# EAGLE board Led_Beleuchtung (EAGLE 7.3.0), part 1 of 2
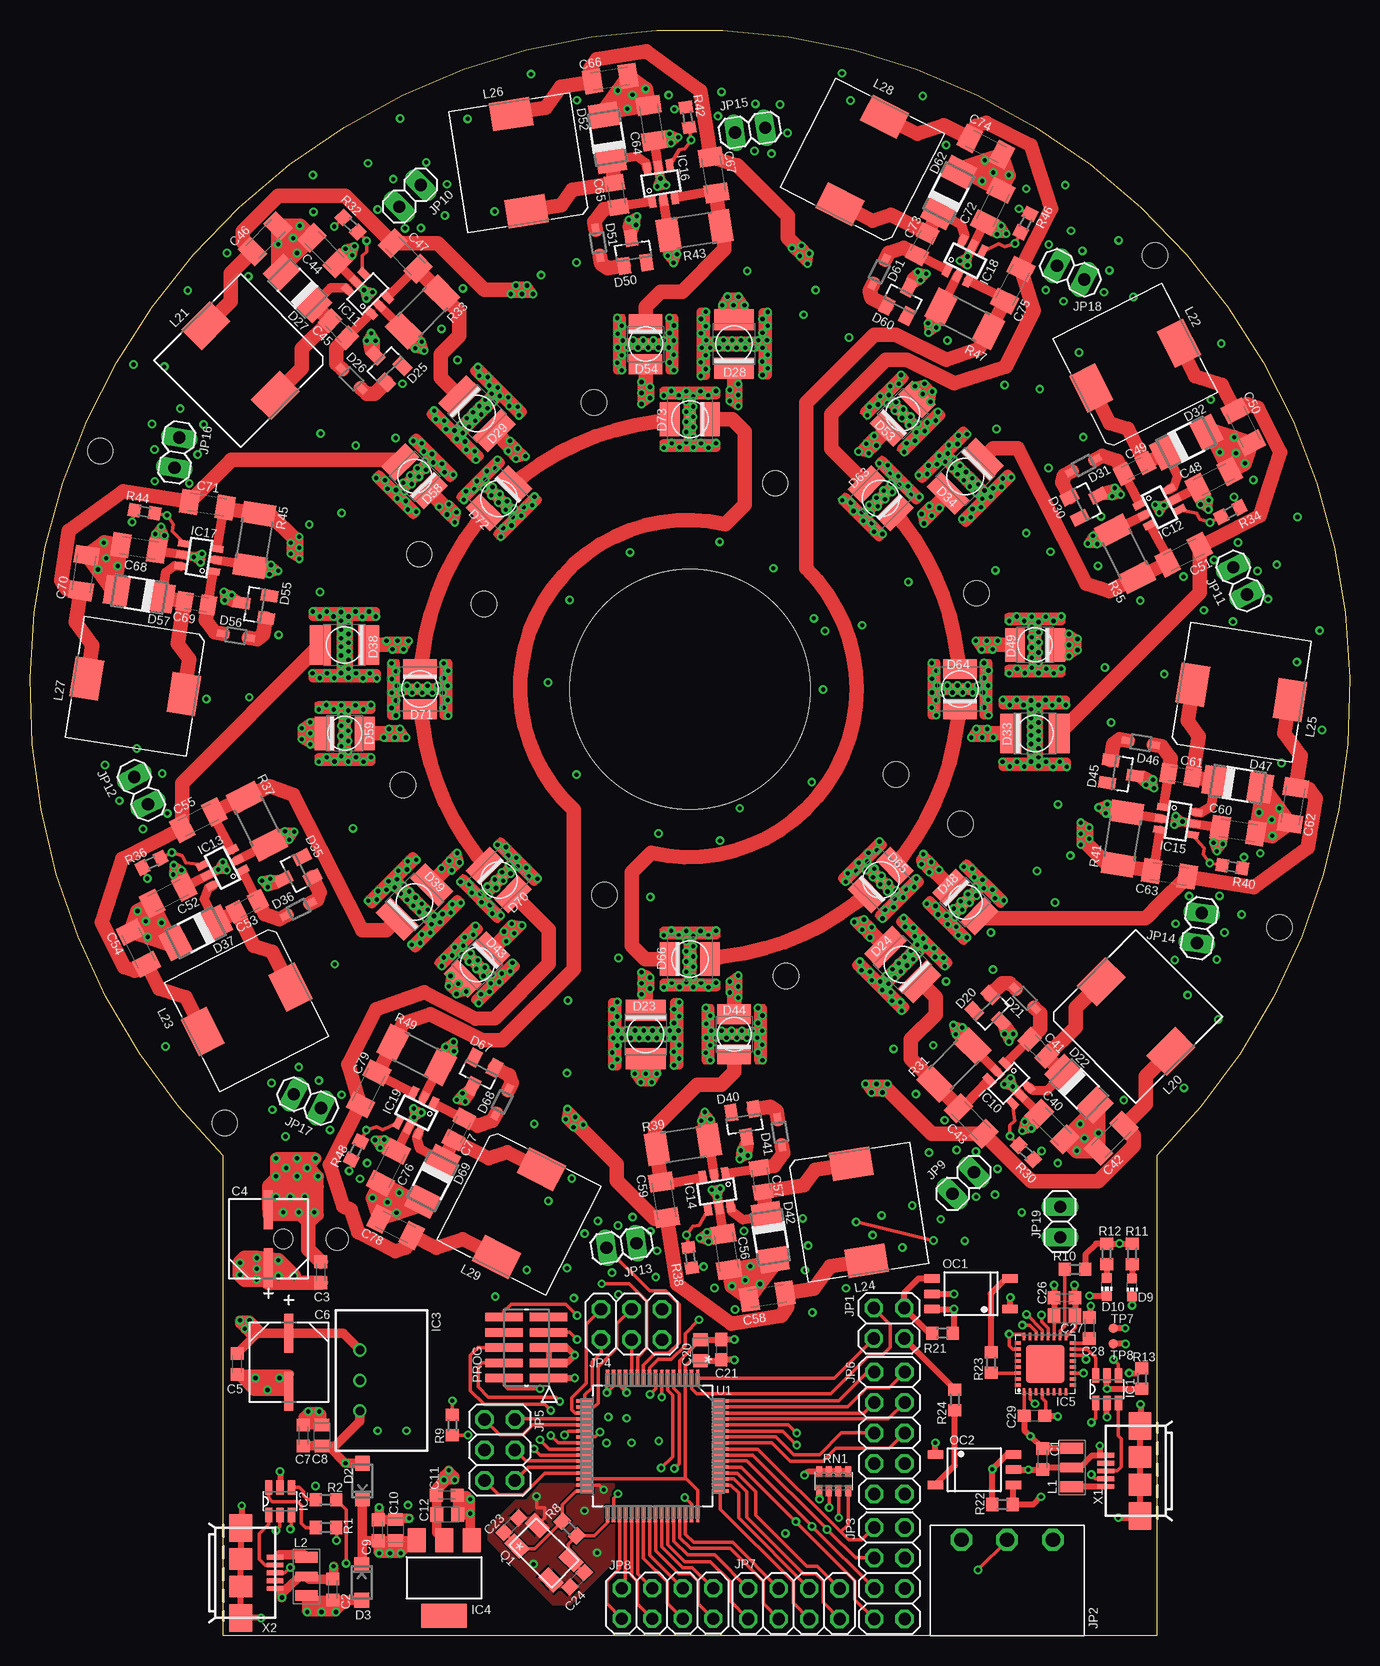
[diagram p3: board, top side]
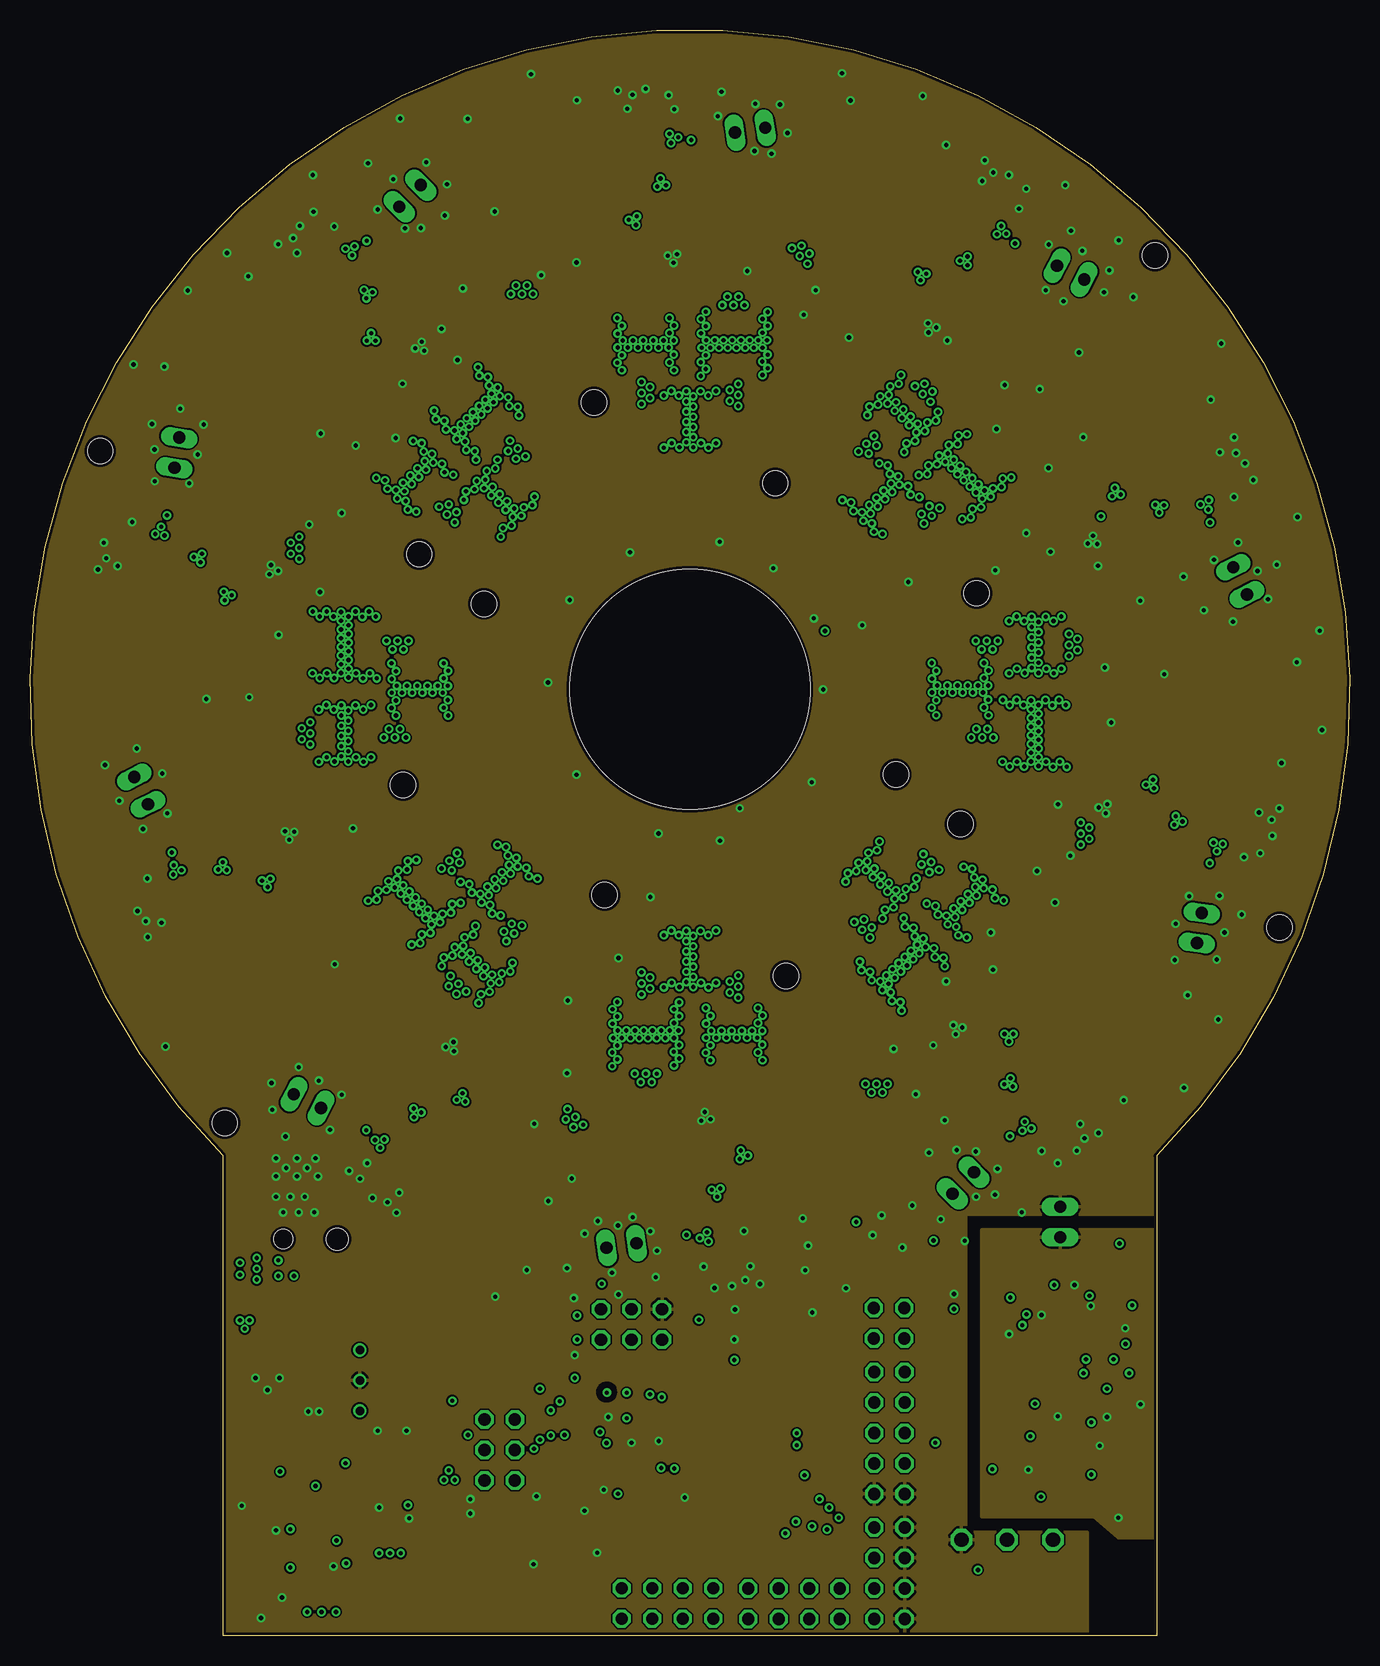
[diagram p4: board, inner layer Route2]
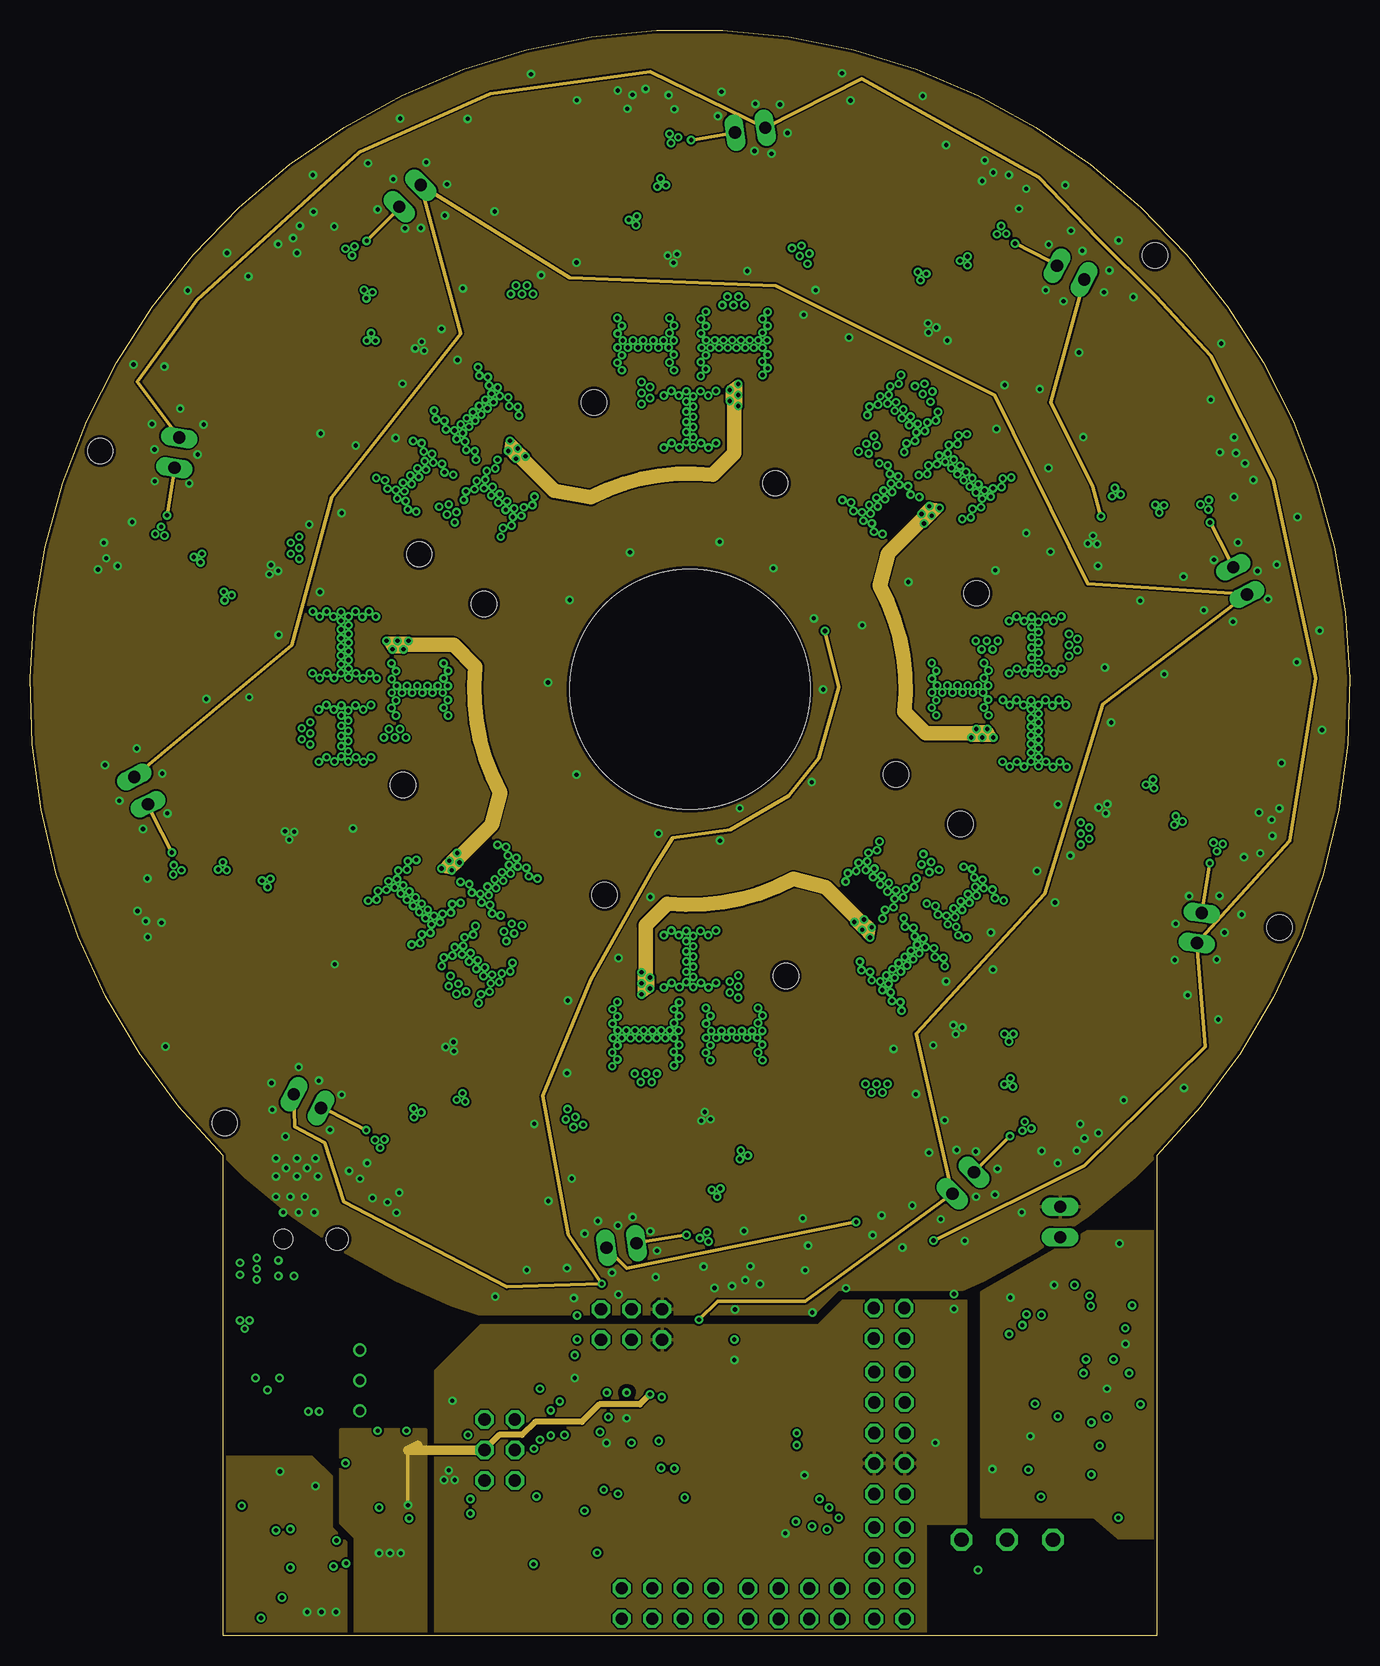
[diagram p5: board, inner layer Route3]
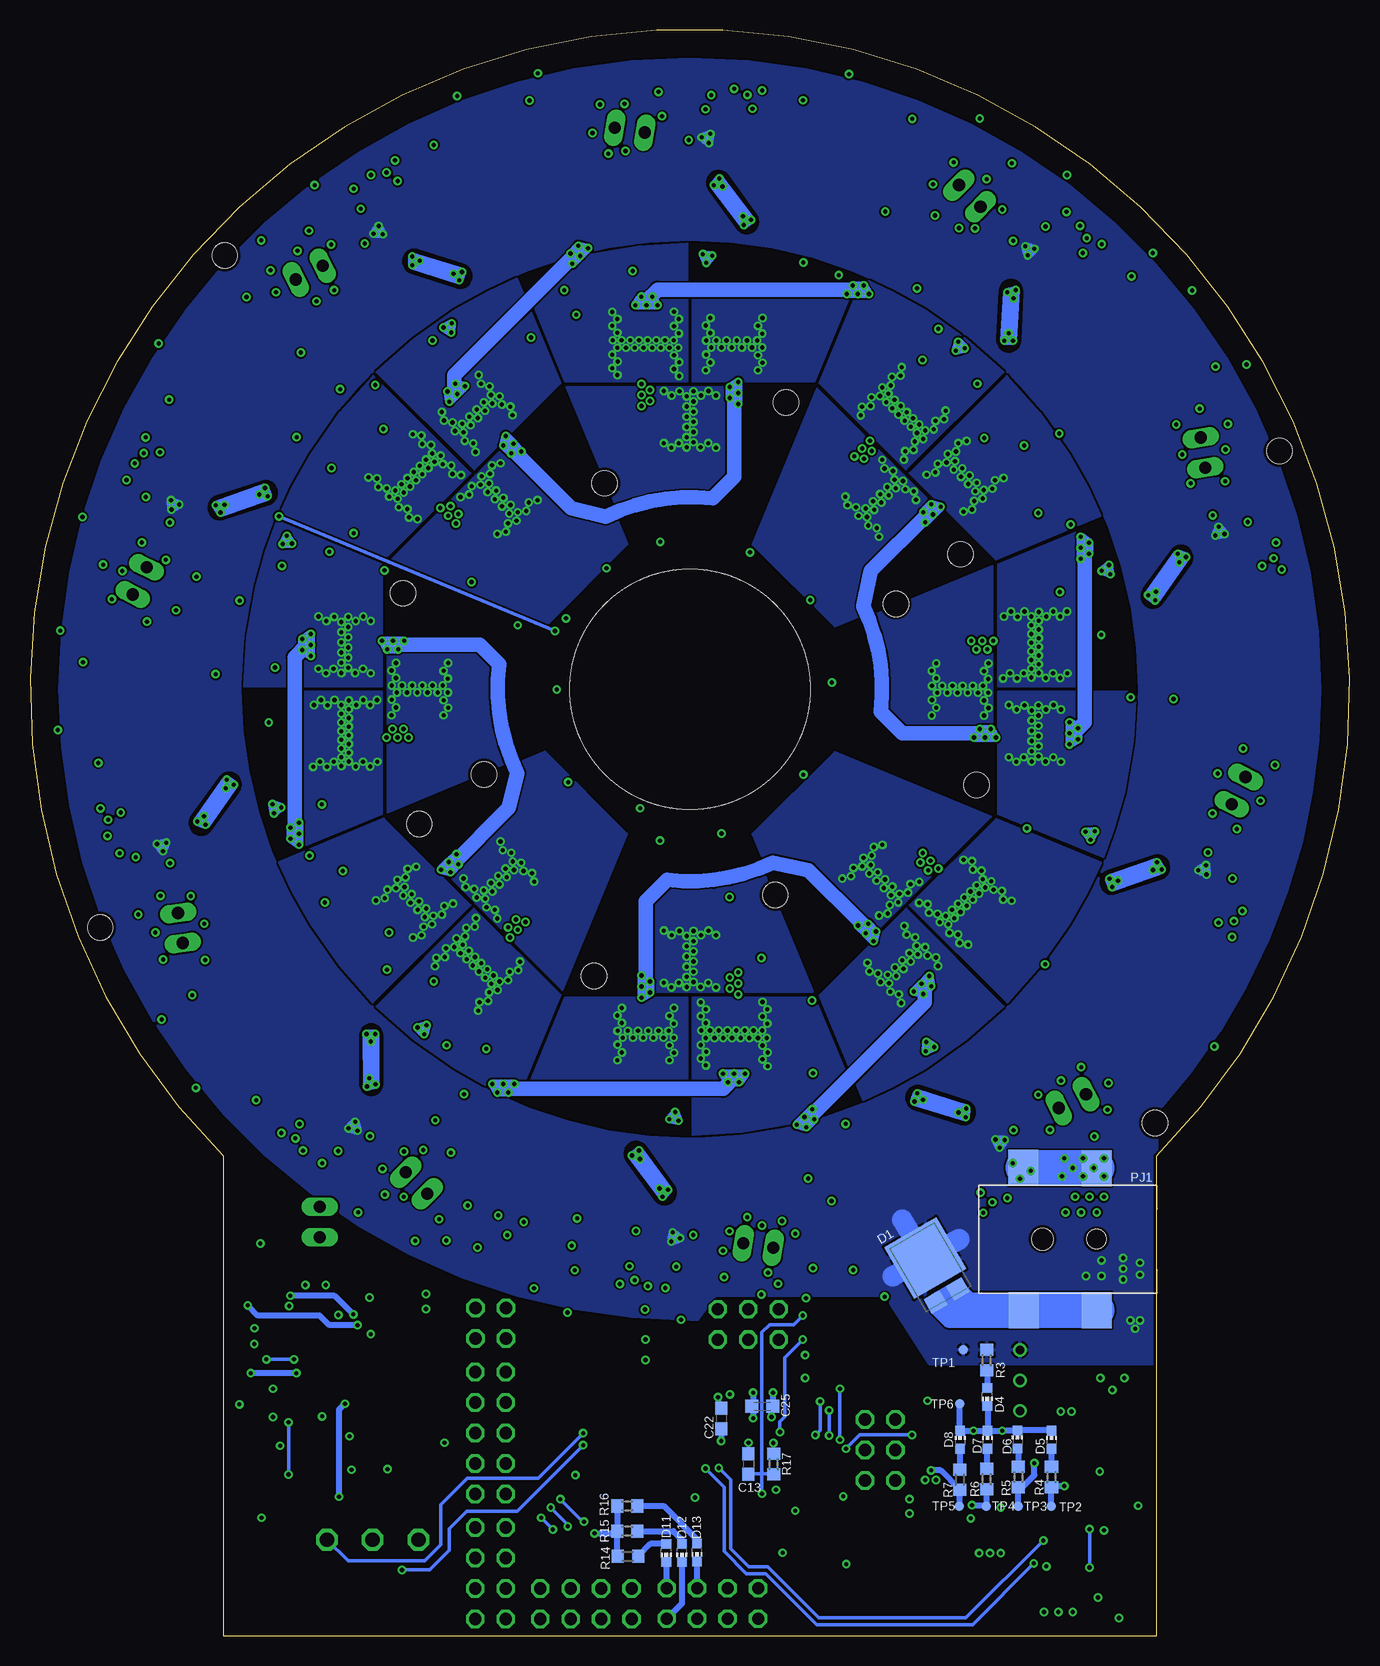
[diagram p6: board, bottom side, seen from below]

Size 109.98 x 133.82 mm. Coordinates in mm from the lower left corner, seen from the top.
Outline: 16.1,0 16.1,39.99 arc-270 93.88,39.99 93.88,0 16.1,0
Copper layers (1+2*3+16): Top 0.018mm / dielectric 0.36mm / Route2 0.035mm / dielectric 0.71mm / Route3 0.035mm / dielectric 0.36mm / Bottom 0.018mm
Design rules "eC_4Layer_PClass6_BaseCopperO18-I35_eCDefault *": minimum track width 0.15mm, minimum drill 0.35mm, track to track 0.15mm, track to pad 0.15mm, pad to pad 0.15mm, via to via 0.15mm, smd to smd 0mil, copper to edge 0.25mm, drill to drill 0.35mm, minimum pad ring 0.175mm, minimum via ring 0.125mm, stop-mask expansion 0mil, vias tented up to drill 0.45mm, thermal gap 0.2mm
Holes 2.1 mm at 62.1,96.05 37.83,85.99 47.88,61.72 72.15,71.78 32.44,90.13 47,102.78 78.89,86.88 77.54,67.64 62.99,54.99 31.09,70.89 5.85,98.74 93.75,115.03 104.13,59.03 16.23,42.74
Holes 20 mm at 54.99,78.88

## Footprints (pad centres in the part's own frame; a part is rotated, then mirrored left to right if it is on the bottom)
C0603K = smd 1.05 x 1.08: 1 -0.875,0; 2 0.875,0
CAPAE660X800N = smd 3.251 x 0.762: 1 -2.413,0; 2 2.413,0
CAPAE660X610N = smd 3.251 x 0.762: 1 -2.413,0; 2 2.413,0
SMC_P = smd 1.05 x 1.2: + -0.875,0; - 0.875,0
C0603 = smd 1.1 x 1: 1 -0.85,0; 2 0.85,0
C1206K = smd 1.5 x 2: 1 -1.5,0; 2 1.5,0
C0805K = smd 1.3 x 1.6: 1 -1,0; 2 1,0
TO-277A = smd 1.5 x 1.4: A1 1.065,-2.705; A2 -1.065,-2.705 | smd 5 x 5: C 0,0.895
SOD-123 = smd 1.25 x 1.22: A 1.475,0; C -1.475,0
CHIP-LED0603 = smd 0.8 x 0.8: A 0,-0.75; C 0,0.75
SOT23 = smd 1 x 1.4: 1 -0.95,-1.1; 2 0.95,-1.1; 3 0,1.1
SOD323 = smd 1 x 0.6: A 1.1,0; C -1.1,0
DO-214AC = smd 2 x 2.4: A 1.9,0; C -1.9,0
LTPL-C034UVH = smd 3.3 x 1.75: A 0,2.025; C 0,-2.025 | smd 1.27 x 0.635: TH 0,0
GW_CSSRM2.PM = smd 2.8 x 1.65: A 0,1.675; C 0,-1.675 | smd 1.27 x 0.635: TH 0,0
SFH_4715 = smd 2.8 x 1.65: A 0,1.675; C 0,-1.675 | smd 1.27 x 0.635: TH 0,0
SOT-23-6L = smd 0.6 x 1.2: 1 -0.95,-1.15; 2 0,-1.15; 3 0.95,-1.15; 4 0.95,1.15; 5 0,1.15; 6 -0.95,1.15
TSR-1 = drill 0.7 pad 1.1: 1 -2.54,0; 2 0,0; 3 2.54,0
SOT223 = smd 1.5 x 2: 1 -2.3,-3.15; 2 0,-3.15; 3 2.3,-3.15 | smd 3.8 x 2: 4 0,3.15
QFN32 = smd 0.6 x 0.3: 1 -2.3,1.75; 2 -2.3,1.25; 3 -2.3,0.75; 4 -2.3,0.25; 5 -2.3,-0.25; 6 -2.3,-0.75; 7 -2.3,-1.25; 8 -2.3,-1.75; 17 2.3,-1.75; 18 2.3,-1.25; 19 2.3,-0.75; 20 2.3,-0.25; 21 2.3,0.25; 22 2.3,0.75; 23 2.3,1.25; 24 2.3,1.75 | smd 0.3 x 0.6: 9 -1.75,-2.3; 10 -1.25,-2.3; 11 -0.75,-2.3; 12 -0.25,-2.3; 13 0.25,-2.3; 14 0.75,-2.3; 15 1.25,-2.3; 16 1.75,-2.3; 25 1.75,2.3; 26 1.25,2.3; 27 0.75,2.3; 28 0.25,2.3; 29 -0.25,2.3; 30 -0.75,2.3; 31 -1.25,2.3; 32 -1.75,2.3 | smd 3.2 x 3.2: EXP 0,0
DDC6_SOT = smd 0.6 x 1.1: 1 -0.95,-1.35; 2 0,-1.35; 3 0.95,-1.35; 4 0.95,1.35; 5 0,1.35; 6 -0.95,1.35
2X02 = drill 1.016 octagon: 1 -1.27,-1.27; 2 -1.27,1.27; 3 1.27,-1.27; 4 1.27,1.27
BCH-381H-3GN = drill 1.2 octagon: 1 3.81,8; 2 0,8; 3 -3.81,8
2X04 = drill 1.016 octagon: 1 -3.81,-1.27; 2 -3.81,1.27; 3 -1.27,-1.27; 4 -1.27,1.27; 5 1.27,-1.27; 6 1.27,1.27; 7 3.81,-1.27; 8 3.81,1.27
2X03 = drill 1.016 octagon: 1 -2.54,-1.27; 2 -2.54,1.27; 3 0,-1.27; 4 0,1.27; 5 2.54,-1.27; 6 2.54,1.27
2X05 = drill 1.016 octagon: 1 -5.08,-1.27; 2 -5.08,1.27; 3 -2.54,-1.27; 4 -2.54,1.27; 5 0,-1.27; 6 0,1.27; 7 2.54,-1.27; 8 2.54,1.27; 9 5.08,-1.27; 10 5.08,1.27
1X02 = drill 1.016 long: 1 -1.27,0; 2 1.27,0
EMIFILTER = smd 0.9 x 1.9: 1 -1.6,0; 3 1.6,0 | smd 0.8 x 1.9: 2 0,0
WE-PDF = smd 3.4 x 2.4: 1 0,4.1; 2 0,-4.1
PC400 = smd 0.7 x 1.3: 1 -1.27,-3.25; 3 1.27,-3.25; 4 1.27,3.25; 5 0,3.25; 6 -1.27,3.25
PJ-002AH-SMT-TR = smd 2.5 x 3: 1.1 5,5.915; 1.2 11.05,5.915; 2 5,-5.915; 3 11.1,-5.965 | hole 1.6: 5,0 | hole 1.8: 9.5,0
SAMTEC_FTS105-01-L-DV = smd 0.711 x 3.124: 1 -2.54,-1.854; 2 -2.54,1.854; 3 -1.27,-1.854; 4 -1.27,1.854; 5 0,-1.854; 6 0,1.854; 7 1.27,-1.854; 8 1.27,1.854; 9 2.54,-1.854; 10 2.54,1.854
ABM3B = smd 1.8 x 1.2: 1 -2,-1.2; 3 2,1.2; GND1 -2,1.2; GND2 2,-1.2
R0603 = smd 1 x 1.1: 1 -0.85,0; 2 0.85,0
R2010 = smd 1.8 x 2.7: 1 -2.2,0; 2 2.2,0
CTS742C083 = smd 0.5 x 0.9: 1 -1.2,-0.8; 2 -0.4,-0.8; 3 0.4,-0.8; 4 1.2,-0.8; 5 1.2,0.8; 6 0.4,0.8; 7 -0.4,0.8; 8 -1.2,0.8
TP08R = smd 0.8 x 0.8: TP 0,0
QFP50P1200X1200X160-64N = smd 1.422 x 0.279: 1 -5.639,3.759; 2 -5.639,3.251; 3 -5.639,2.743; 4 -5.639,2.261; 5 -5.639,1.753; 6 -5.639,1.245; 7 -5.639,0.762; 8 -5.639,0.254; 9 -5.639,-0.254; 10 -5.639,-0.762; 11 -5.639,-1.245; 12 -5.639,-1.753; 13 -5.639,-2.261; 14 -5.639,-2.743; 15 -5.639,-3.251; 16 -5.639,-3.759; 33 5.639,-3.759; 34 5.639,-3.251; 35 5.639,-2.743; 36 5.639,-2.261; 37 5.639,-1.753; 38 5.639,-1.245; 39 5.639,-0.762; 40 5.639,-0.254; 41 5.639,0.254; 42 5.639,0.762; 43 5.639,1.245; 44 5.639,1.753; 45 5.639,2.261; 46 5.639,2.743; 47 5.639,3.251; 48 5.639,3.759 | smd 0.279 x 1.422: 17 -3.759,-5.639; 18 -3.251,-5.639; 19 -2.743,-5.639; 20 -2.261,-5.639; 21 -1.753,-5.639; 22 -1.245,-5.639; 23 -0.762,-5.639; 24 -0.254,-5.639; 25 0.254,-5.639; 26 0.762,-5.639; 27 1.245,-5.639; 28 1.753,-5.639; 29 2.261,-5.639; 30 2.743,-5.639; 31 3.251,-5.639; 32 3.759,-5.639; 49 3.759,5.639; 50 3.251,5.639; 51 2.743,5.639; 52 2.261,5.639; 53 1.753,5.639; 54 1.245,5.639; 55 0.762,5.639; 56 0.254,5.639; 57 -0.254,5.639; 58 -0.762,5.639; 59 -1.245,5.639; 60 -1.753,5.639; 61 -2.261,5.639; 62 -2.743,5.639; 63 -3.251,5.639; 64 -3.759,5.639
MICRO-USB = smd 0.4 x 1.4: 1 -1.3,2.85; 2 -0.65,2.85; 3 0,2.85; 4 0.65,2.85; 5 1.3,2.85 | smd 2.3 x 1.9: GND1 -3.75,0; GND2 3.75,0 | smd 1.8 x 1.9: GND3 -1.15,0; GND4 1.15,0

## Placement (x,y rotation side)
C1  100nF  [C0603K]  84.38,14.73 90 top
C2  100nF  [C0603K]  25.23,3.85 270 top
C3  100nF  [C0603K]  24.23,30.29 270 top
C4  100UF  [CAPAE660X800N]  19.87,33.09 90 top
C5  100nF  [C0603K]  17.26,22.66 90 top
C6  22uF  [CAPAE660X610N]  21.58,22.79 270 top
C7  100nF  [C0603K]  22.78,16.68 270 top
C8  10uF  [SMC_P]  24.33,16.7 90 top
C9  100nF  [C0603K]  29.01,8.79 270 top
C10  10uF  [SMC_P]  30.46,8.8 90 top
C11  100nF  [C0603K]  34.73,11.72 180 top
C12  10uF  [SMC_P]  34.77,10.1 0 top
C13  100nF  [C0603]  50.12,14.31 270 bottom
C20  10uF  [SMC_P]  55.89,23.8 90 top
C21  100nF  [C0603]  57.61,23.85 270 top
C22  2.2uF  [C0603]  52.39,18.1 270 bottom
C23  22pF  [C0603]  40.1,9.21 45 top
C24  22pF  [C0603]  45.6,4.67 225 top
C25  100nF  [C0603K]  48.96,19.12 180 bottom
C26  100nF  [C0603K]  86.21,28.17 180 top
C27  4.7uF  [SMC_P]  86.22,26.7 0 top
C28  100nF  [C0603K]  88.28,25.66 270 top
C29  100nF  [C0603]  83.71,18.32 180 top
C40  10uF  [C1206K]  85.16,42.45 135 top
C41  0.01uF  [C0805K]  83.99,49 315 top
C42  1uF  [C1206K]  90.1,41.46 45 top
C43  1uF  [C1206K]  78.43,42.89 135 top
C44  10uF  [C1206K]  24.55,115.43 315 top
C45  0.01uF  [C0805K]  25.72,108.88 135 top
C46  1uF  [C1206K]  19.61,116.42 225 top
C47  1uF  [C1206K]  31.28,114.99 315 top
C48  10uF  [C1206K]  98.65,96.36 207 top
C49  0.01uF  [C0805K]  92.05,97.27 27 top
C50  1uF  [C1206K]  101.11,100.75 117 top
C51  1uF  [C1206K]  96.14,90.09 207 top
C52  10uF  [C1206K]  11.51,61.7 27 top
C53  0.01uF  [C0805K]  18.1,60.79 207 top
C54  1uF  [C1206K]  9.04,57.31 297 top
C55  1uF  [C1206K]  14.02,67.97 27 top
C56  10uF  [C1206K]  58.02,32 99 top
C57  0.01uF  [C0805K]  60.93,37.99 279 top
C58  1uF  [C1206K]  61.44,28.3 9 top
C59  1uF  [C1206K]  52.84,36.32 99 top
C60  10uF  [C1206K]  100.67,67.1 171 top
C61  0.01uF  [C0805K]  95.87,71.71 351 top
C62  1uF  [C1206K]  105.24,69.2 81 top
C63  1uF  [C1206K]  94.96,63.5 171 top
C64  10uF  [C1206K]  51.78,126.05 279 top
C65  0.01uF  [C0805K]  48.88,120.06 99 top
C66  1uF  [C1206K]  48.37,129.76 189 top
C67  1uF  [C1206K]  56.97,121.73 279 top
C68  10uF  [C1206K]  9.06,90.66 351 top
C69  0.01uF  [C0805K]  13.86,86.04 171 top
C70  1uF  [C1206K]  4.49,88.56 261 top
C71  1uF  [C1206K]  14.78,94.25 351 top
C72  10uF  [C1206K]  80.24,119.11 243 top
C73  0.01uF  [C0805K]  74.37,115.97 63 top
C74  1uF  [C1206K]  79.65,124.11 153 top
C75  1uF  [C1206K]  81.89,112.56 243 top
C76  10uF  [C1206K]  29.87,39.06 63 top
C77  0.01uF  [C0805K]  35.75,42.19 243 top
C78  1uF  [C1206K]  30.46,34.05 333 top
C79  1uF  [C1206K]  28.22,45.6 63 top
D1  AS3PM  [TO-277A]  34.95,30.71 30 bottom
D2  MBR120VLSFT1  [SOD-123]  27.7,12.91 90 top
D3  MBR120VLSFT1  [SOD-123]  27.65,4.43 270 top
D4  gn  [CHIP-LED0603]  30.21,19.91 180 bottom
D5  gn  [CHIP-LED0603]  24.86,16.34 0 bottom
D6  gn  [CHIP-LED0603]  27.7,16.36 0 bottom
D7  gn  [CHIP-LED0603]  30.19,16.34 0 bottom
D8  gn  [CHIP-LED0603]  32.47,16.34 0 bottom
D9  gn  [CHIP-LED0603]  91.85,29.02 180 top
D10  yw  [CHIP-LED0603]  89.73,29.07 180 top
D11  gn  [CHIP-LED0603]  56.97,6.9 180 bottom
D12  rd  [CHIP-LED0603]  55.67,6.9 180 bottom
D13  yw  [CHIP-LED0603]  54.4,6.94 180 bottom
D20  8V2  [SOT23]  80.13,51.96 225 top
D21  CMDSH-3  [SOD323]  82.92,53.13 135 top
D22  SS13  [DO-214AC]  87.41,45.59 315 top
D23  LTPL-C034UVH  [LTPL-C034UVH]  51.31,50.12 180 top
D24  LTPL-C034UVH  [LTPL-C034UVH]  72.72,55.94 45 top
D25  8V2  [SOT23]  29.58,105.92 45 top
D26  CMDSH-3  [SOD323]  26.79,104.75 315 top
D27  SS13  [DO-214AC]  22.3,112.29 135 top
D28  LTPL-C034UVH  [LTPL-C034UVH]  58.67,107.65 0 top
D29  LTPL-C034UVH  [LTPL-C034UVH]  37.25,101.84 225 top
D30  8V2  [SOT23]  88.04,94.52 297 top
D31  CMDSH-3  [SOD323]  87.79,97.52 207 top
D32  SS13  [DO-214AC]  96.35,99.46 27 top
D33  LTPL-C034UVH  [LTPL-C034UVH]  83.75,75.2 270 top
D34  LTPL-C034UVH  [LTPL-C034UVH]  77.94,96.63 135 top
D35  8V2  [SOT23]  22.12,63.54 117 top
D36  CMDSH-3  [SOD323]  22.37,60.53 27 top
D37  SS13  [DO-214AC]  13.8,58.59 207 top
D38  LTPL-C034UVH  [LTPL-C034UVH]  26.22,82.58 90 top
D39  LTPL-C034UVH  [LTPL-C034UVH]  32.04,61.16 315 top
D40  8V2  [SOT23]  59.55,42.65 189 top
D41  CMDSH-3  [SOD323]  62.49,41.96 99 top
D42  SS13  [DO-214AC]  61.69,33.22 279 top
D43  GW_CSSRM2.PM  [GW_CSSRM2.PM]  37.26,55.94 135 top
D44  GW_CSSRM2.PM  [GW_CSSRM2.PM]  58.68,50.12 0 top
D45  8V2  [SOT23]  91,71.84 261 top
D46  CMDSH-3  [SOD323]  92.57,74.42 171 top
D47  SS13  [DO-214AC]  100.64,70.96 351 top
D48  GW_CSSRM2.PM  [GW_CSSRM2.PM]  77.94,61.15 225 top
D49  GW_CSSRM2.PM  [GW_CSSRM2.PM]  83.75,82.58 90 top
D50  8V2  [SOT23]  50.26,115.4 9 top
D51  CMDSH-3  [SOD323]  47.32,116.09 279 top
D52  SS13  [DO-214AC]  48.12,124.83 99 top
D53  GW_CSSRM2.PM  [GW_CSSRM2.PM]  72.72,101.84 315 top
D54  GW_CSSRM2.PM  [GW_CSSRM2.PM]  51.31,107.65 180 top
D55  8V2  [SOT23]  18.73,85.91 81 top
D56  CMDSH-3  [SOD323]  17.16,83.33 351 top
D57  SS13  [DO-214AC]  9.09,86.8 171 top
D58  GW_CSSRM2.PM  [GW_CSSRM2.PM]  32.05,96.62 45 top
D59  GW_CSSRM2.PM  [GW_CSSRM2.PM]  26.22,75.2 270 top
D60  8V2  [SOT23]  72.74,111.38 333 top
D61  CMDSH-3  [SOD323]  70.77,113.67 243 top
D62  SS13  [DO-214AC]  76.56,120.27 63 top
D63  SFH_4715  [SFH_4715]  70.9,94.79 45 top
D64  SFH_4715  [SFH_4715]  77.49,78.9 0 top
D65  SFH_4715  [SFH_4715]  70.9,62.98 315 top
D66  SFH_4715  [SFH_4715]  54.99,56.39 270 top
D67  8V2  [SOT23]  37.37,46.78 153 top
D68  CMDSH-3  [SOD323]  39.34,44.49 63 top
D69  SS13  [DO-214AC]  33.56,37.89 243 top
D70  SFH_4715  [SFH_4715]  39.08,62.98 225 top
D71  SFH_4715  [SFH_4715]  32.49,78.88 180 top
D72  SFH_4715  [SFH_4715]  39.08,94.79 135 top
D73  SFH_4715  [SFH_4715]  54.99,101.38 90 top
IC1  USBLC6-2  [SOT-23-6L]  89.75,20.55 0 top
IC2  USBLC6-2  [SOT-23-6L]  20.84,11.21 0 top
IC3  TSR-12450  [TSR-1]  27.49,21.28 270 top
IC4  NCP1117ST33T3G  [SOT223]  34.51,4.83 180 top
IC5  FT232RQ  [QFN32]  84.6,22.64 90 top
IC10  LM3405A  [DDC6_SOT]  81.57,46.04 225 top
IC11  LM3405A  [DDC6_SOT]  28.14,111.84 45 top
IC12  LM3405A  [DDC6_SOT]  94.12,94.05 297 top
IC13  LM3405A  [DDC6_SOT]  16.04,64.01 117 top
IC14  LM3405A  [DDC6_SOT]  57.23,37.02 189 top
IC15  LM3405A  [DDC6_SOT]  95.65,67.89 261 top
IC16  LM3405A  [DDC6_SOT]  52.58,121.04 9 top
IC17  LM3405A  [DDC6_SOT]  14.08,89.86 81 top
IC18  LM3405A  [DDC6_SOT]  77.93,114.58 333 top
IC19  LM3405A  [DDC6_SOT]  32.18,43.58 153 top
JP1  [2X02]  71.59,26.04 90 top
JP2  [BCH-381H-3GN]  81.43,0 0 top
JP3  [2X04]  71.62,5.22 270 top
JP4  [2X03]  50.13,25.95 180 top
JP5  [2X03]  39.14,15.48 270 top
JP6  [2X05]  71.62,16.9 270 top
JP7  [2X04]  63.66,2.67 180 top
JP8  [2X04]  53.12,2.69 180 top
JP9  [1X02]  77.77,37.74 45 top
JP10  [1X02]  31.68,119.99 225 top
JP11  [1X02]  100.84,87.91 117 top
JP12  [1X02]  9.26,70.43 297 top
JP13  [1X02]  49.29,32.52 9 top
JP14  [1X02]  97.45,58.98 81 top
JP15  [1X02]  60.01,125.47 189 top
JP16  [1X02]  12.23,98.6 261 top
JP17  [1X02]  23.12,44.55 333 top
JP18  [1X02]  86.71,113.6 153 top
JP19  [1X02]  85.84,34.48 270 top
L1  NFE31  [EMIFILTER]  86.82,14.02 90 top
L2  NFE31  [EMIFILTER]  23.05,4.95 270 top
L20  22uH  [WE-PDF]  92.17,51.61 45 top
L21  22uH  [WE-PDF]  17.54,106.27 225 top
L22  22uH  [WE-PDF]  92.1,105.85 117 top
L23  22uH  [WE-PDF]  18.06,52.21 297 top
L24  13uH  [WE-PDF]  69.07,35.29 9 top
L25  13uH  [WE-PDF]  100.95,78.62 81 top
L26  13uH  [WE-PDF]  40.73,122.76 189 top
L27  13uH  [WE-PDF]  8.78,79.13 261 top
L28  11uH  [WE-PDF]  69.36,122.94 153 top
L29  11uH  [WE-PDF]  40.75,35.22 333 top
OC1  PC400  [PC400]  78.42,28.5 90 top
OC2  PC400  [PC400]  78.7,13.84 270 top
PJ1  PJ-002AH-SMT-TR  [PJ-002AH-SMT-TR]  16.1,33.06 180 bottom
PROG  FTS105-01-L-DV  [SAMTEC_FTS105-01-L-DV]  41.36,24.01 90 top
Q1  ABM3B4PIN  [ABM3B]  42.84,6.92 315 top
R1  33R  [R0603]  24.65,9.02 0 top
R2  33R  [R0603]  24.65,11.34 0 top
R3  8k2  [R0603]  30.26,22.97 90 bottom
R4  1k5  [R0603]  24.87,13.22 270 bottom
R5  1k5  [R0603]  27.63,13.23 270 bottom
R6  1k5  [R0603]  30.27,13.05 270 bottom
R7  620R  [R0603]  32.5,13 270 bottom
R8  1M  [R0603]  44.96,8.95 135 top
R9  10k  [R0603]  35.19,17.55 270 top
R10  10k  [R0603]  87.09,30.53 0 top
R11  1k8  [R0603]  91.85,31.83 270 top
R12  2k2  [R0603]  89.73,31.83 90 top
R13  10k  [R0603]  92.65,21.43 270 top
R14  620R  [R0603]  60.17,6.62 180 bottom
R15  1k  [R0603]  60.22,8.72 180 bottom
R16  1k  [R0603]  60.22,10.82 180 bottom
R17  10k  [R0603]  48.02,14.31 270 bottom
R21  4k7  [R0603]  76.03,25.22 180 top
R22  4k7  [R0603]  81.04,10.94 0 top
R23  1k  [R0603]  80.1,22.77 270 top
R24  1k  [R0603]  77.07,19.66 270 top
R30  39k  [R0603]  83.01,40.29 135 top
R31  0R4  [R2010]  76.99,47.56 45 top
R32  39k  [R0603]  26.7,117.59 315 top
R33  0R4  [R2010]  32.72,110.32 225 top
R34  39k  [R0603]  100.03,93.64 207 top
R35  0R4  [R2010]  91.25,90.17 117 top
R36  39k  [R0603]  10.13,64.42 27 top
R37  0R4  [R2010]  18.9,67.89 297 top
R38  39k  [R0603]  55.01,31.52 99 top
R39  0R3  [R2010]  54.42,40.94 9 top
R40  39k  [R0603]  100.19,64.09 171 top
R41  0R3  [R2010]  91.05,66.43 81 top
R42  39k  [R0603]  54.79,126.53 279 top
R43  0R3  [R2010]  55.39,117.11 189 top
R44  39k  [R0603]  9.54,93.67 351 top
R45  0R3  [R2010]  18.68,91.32 261 top
R46  20k  [R0603]  82.96,117.72 243 top
R47  0R25  [R2010]  77.9,109.75 153 top
R48  20k  [R0603]  27.16,40.44 63 top
R49  0R25  [R2010]  32.22,48.41 333 top
RN1  10k  [CTS742C083]  66.97,12.9 0 top
TP1  +12V  [TP08R]  32.21,23.85 180 bottom
TP2  +5V_USB  [TP08R]  24.86,10.8 0 bottom
TP3  +5V_Reg  [TP08R]  27.64,10.8 0 bottom
TP4  +5V  [TP08R]  30.29,10.8 0 bottom
TP5  +3V3  [TP08R]  32.54,10.8 0 bottom
TP6  GND  [TP08R]  32.49,19.35 0 bottom
TP7  GND  [TP08R]  90.26,25.63 270 top
TP8  +5V  [TP08R]  90.28,24.32 90 top
U1  MKL26Z256VLH4  [QFP50P1200X1200X160-64N]  51.88,15.82 270 top
X1  MICRO_USB  [MICRO-USB]  92.5,13.74 90 top
X2  MICRO_USB  [MICRO-USB]  17.57,5.24 270 top

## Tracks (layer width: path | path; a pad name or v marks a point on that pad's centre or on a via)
3V3OUT_FT232
  Top 0.3: IC5.16 88.19,24.39 arc90 C28.2
+3V3  (via drill 0.35 pad 0.7)
  Top 0.3: U1.13 49.62,20.36 | U1.14 49.14,20.85 v49.72,20.26 | v35.19,19.58 R9.1 | U1.3 54.62,22.52 55.04,22.93 55.88,22.93 C20.+ | 54.64,21.44 U1.3 | U1.30 54.59,13.07 | 54.59,13.07 54.7,13.07 55.64,12.13 U1.48 | U1.3 54.62,13.11 54.59,13.07
  Top 0.305: 49.62,20.36 v49.72,20.26
  Top 0.5: 33.89,12.38 33.89,12.28 33.89,11.58 | RN1.5 RN1.6 RN1.7 RN1.8 64.86,13.7 v64.54,13.38 | PROG.1 v45.39,21.48 | OC2.1 v75.44,16.08 | OC1.6 v76.98,27.23 v76.99,27.23 76.99,25.34 R21.1 | C20.+ 57.54,22.92 C21.2 57.63,22.98 v58.69,22.98
  Top 0.8: IC4.2 33.9,8.59 C12.+ 33.9,11.68 C11.2 33.99,11.85 33.99,12.18 34.79,12.98 v35.39,12.98 35.39,13.28 v34.89,13.78 34.49,13.38 v34.49,12.98 33.89,12.38 | 33.89,12.28 34.99,13.38
  Bottom 0.3: 49.6,19.33 C25.2 | 49.72,19.03 C25.2 | 49.72,19.23 C25.2 | v48.04,16.06 48.04,15.18 R17.1
  Bottom 0.5: 49.72,19.03 v49.72,18.13 | v49.72,20.26 49.72,19.23 | TP5.TP 32.5,10.84 R7.2 32.5,12.19 34.09,13.78 v34.89,13.78 | R14.2 61.07,6.67 R15.2 | R15.2 R16.2 61.07,10.86 | v62.94,8.53 61.25,8.53 R15.2
  pour Route3: 74.59,-1.32 74.59,9.38 77.99,9.38 77.99,27.93 67.74,27.93 65.69,25.88 37.59,25.88 33.79,22.08 33.79,-1.32
+5V  (via drill 0.35 pad 0.7)
  Top 0.3: U1.8 52.14,20.6 v51.66,20.12
  Top 0.8: D2.C 27.7,8.08 | 27.7,8.08 27.7,5.95 D3.C | C9.2 27.86,7.92 27.7,8.08 | C9.2 C10.+ 32.16,7.93 IC4.3 | C9.2 29.01,6.97 v29.09,6.88 v29.99,6.88 v30.89,6.88 31.39,7.38 | 31.69,7.68 31.39,7.38 | 31.39,7.38 29.49,7.38
  Route3 0.3: v31.49,10.88 31.49,15.08 32.29,15.88
  Route3 0.5: v51.66,20.12 50.82,19.28 47.44,19.28 45.99,17.83 42.09,17.83 40.99,16.73 39.09,16.73 37.87,15.51 JP5.3
  Route3 0.8: JP5.3 31.49,15.48 32.29,15.88
  Bottom 0.5: R6.2 30.27,10.82 TP4.TP 30.38,10.88 v31.49,10.88
  pour Route3: 27.09,-0.92 32.99,-0.92 32.99,17.18 25.89,17.18 25.89,9.38 27.09,8.18
+5V_REGLER  (via drill 0.35 pad 0.7)
  Top 0.8: IC3.3 27.49,17.88 25.39,15.78 24.89,15.78 | 24.89,15.78 24.37,15.78 C8.+ 22.8,15.83 C7.2 | D2.A 26.39,14.39 v26.29,14.39 24.89,15.78
  Bottom 0.5: TP3.TP 27.63,10.81 R5.2 27.3,12.38 26.29,13.38 v26.29,14.38 v26.29,14.39
+5V_USB  (via drill 0.35 pad 0.7)
  Top 0.3: IC5.19 C27.+ | IC5.1 82.85,18.33 C29.2
  Top 0.5: IC1.5 89.74,21.69 v89.74,20.58 v89.75,20.58 R13.2 | v91.3,24.32 TP8.TP | L1.3 84.39,15.62 C1.2 v83.36,16.63 | C27.+ 85.35,28.46 C26.2 85.34,28.49 v85.34,29.23 | R11.1 v90.79,32.68 R12.2 88.84,32.68 87.94,31.78 R10.2 | C29.2 82.86,17.13 v83.36,16.63 | v83.36,16.63 | R22.1 v80.19,13.88 81.42,15.11 OC2.6 | OC1.1 81.69,27.25 v81.69,28.18
  pour Route3: 79.29,9.93 79.29,28.63 88.09,33.68 94.99,33.68 94.99,8.18 90.69,8.18 88.64,9.93
+5V_USB_SUP  (via drill 0.35 pad 0.7)
  Top 0.5: v20.84,13.68 IC2.5
  Top 0.8: D3.A 25.25,2.96 C2.2 23.42,2.98 L2.3 23.05,2.03 v23.09,1.98 v24.29,1.98 v25.49,1.98 25.99,2.48 | 26.39,2.88 25.99,2.48 | 25.99,2.48 23.29,2.48
  Bottom 0.5: TP2.TP R4.2 24.75,12.48 v23.79,12.48
  pour Route3: 15.09,14.88 23.49,14.88 25.09,13.28 25.09,8.98 26.29,7.78 26.29,-0.92 15.09,-0.92
+12V  (via drill 0.35 pad 0.7)
  Top 0.7: v26.29,115.58 v27.04,115.78 v26.84,115.03 | v26.29,115.58 v26.84,115.03 | v26.29,115.58 25.61,114.9 C44.2 | v26.84,115.03 26.19,114.38 25.59,114.38 | v10.44,91.82 v10.93,92.42 v11.21,91.69 | v10.44,91.82 v11.21,91.69 | v53.29,125.16 v54.02,124.88 v53.41,124.39 | v53.29,125.16 v53.41,124.39 | v80.93,117.49 v81.35,116.84 v80.58,116.8 | v80.93,117.49 v80.58,116.8 | v98.24,94.63 v98.2,93.86 v97.55,94.28 | v98.24,94.63 v97.55,94.28 | v99.4,65.98 v98.91,65.37 v98.63,66.1 | v99.4,65.98 v98.63,66.1 | v83.44,42.28 v82.69,42.08 v82.89,42.83 | v83.44,42.28 v82.89,42.83 | v56.55,32.86 v55.82,33.14 v56.42,33.63 | v56.55,32.86 v56.42,33.63 | v29.18,40.67 v28.76,41.32 v29.53,41.36 | v29.18,40.67 v29.53,41.36 | v11.94,63.44 v11.98,64.22 v12.63,63.8 | v11.94,63.44 v12.63,63.8 | v11.94,63.44 12.34,62.63 | v12.63,63.8 13.14,62.83 C52.2 12.29,63.58 | v10.44,91.82 10.29,90.93 C68.2 | v11.21,91.69 11.04,90.68 10.74,91.43 | v53.41,124.39 52.63,124.27 C64.2 | v53.29,125.16 52.49,125.03 53.09,124.73 | v80.58,116.8 79.84,117.18 C72.2 | v80.93,117.49 79.94,117.98 80.59,117.23 | v97.55,94.28 97.09,95.13 C48.2 | v98.24,94.63 97.74,95.53 97.84,94.73 | v98.63,66.1 98.74,66.78 C60.2 | v99.4,65.98 99.54,67.13 99.09,66.38 | v82.89,42.83 83.44,43.38 C40.2 | v83.44,42.28 84.14,42.98 83.39,42.73 | v56.42,33.63 57.34,33.78 56.69,33.23 | v56.55,32.86 57.49,33.03 C56.2 | v29.53,41.36 30.24,40.98 C76.2 | v29.18,40.67 30.04,40.23 29.64,40.83 | v28.79,107.93 v28.43,108.55 v28.07,107.93 | v28.07,107.93 v28.79,107.93 | v16.81,86.72 v16.15,87.01 v16.22,86.29 | v16.22,86.29 v16.81,86.72 | v50.49,117.57 v50.57,118.28 v49.91,117.99 | v49.91,117.99 v50.49,117.57
  Top 0.7: v74.22,112.96 v74.7,113.5 v73.99,113.66 | v73.99,113.66 v74.22,112.96 | v36.05,45.21 v35.56,44.67 v36.27,44.52 | v36.27,44.52 v36.05,45.21 | v20.03,63.08 v19.33,62.93 v19.81,62.39 | v19.81,62.39 v20.03,63.08 | v90.18,94.96 v90.88,95.11 v90.4,95.65 | v90.4,95.65 v90.18,94.96 | v93,70.92 v93.66,70.63 v93.59,71.35 | v93.59,71.35 v93,70.92 | v81.22,50.15 v81.58,49.53 v81.94,50.15 | v81.94,50.15 v81.22,50.15 | v59.23,40.45 v59.16,39.73 v59.82,40.02 | v59.82,40.02 v59.23,40.45 | D60.3 v74.22,112.96 | v73.99,113.66 73.49,113.23 73.29,112.78 | v50.49,117.57 D50.3 | v49.91,117.99 49.74,117.43 49.89,116.78 | v28.79,107.93 D25.3 | v28.07,107.93 28.24,107.03 28.74,106.63 | v16.81,86.72 D55.3 | v16.22,86.29 16.89,86.03 17.54,85.98 | v20.03,63.08 D35.3 | v19.81,62.39 20.59,62.58 20.99,62.93 | v36.05,45.21 D67.3 | v36.27,44.52 36.79,45.28 36.79,45.53 | v59.23,40.45 D40.3 | v59.82,40.02 59.99,40.98 59.64,41.53 | v81.22,50.15 D20.3 | v81.94,50.15 81.49,50.83 81.09,51.13 | v93,70.92 D45.3 | v93.59,71.35 92.79,71.73 92.19,71.78 | v90.18,94.96 D30.3 | v90.4,95.65 89.49,95.43 89.04,95.08 | v77.5,114.58 v78.13,114.93 v78.12,114.21 v77.5,114.58 | v93.78,94.25 v94.5,94.21 v94.1,93.6 v93.78,94.25 | v28.03,111.45 v27.84,112.15 v28.54,111.96 v28.03,111.45 | v14.21,89.45 v13.65,89.91 v14.33,90.17 v14.21,89.45 | v16.4,63.82 v15.68,63.85 v16.07,64.46 v16.4,63.82 | v95.48,68.3 v96.04,67.85 v95.36,67.59 v95.48,68.3 | v81.71,46.46 v81.9,45.77 v81.2,45.96 v81.71,46.46 | v32.61,43.61 v32.01,43.21 v31.97,43.94 v32.61,43.61 | v57.53,37.27 v57.27,36.6 v56.81,37.16 v57.53,37.27 | v52.28,120.77 v52.54,121.45 v53,120.88 v52.28,120.77
  Top 0.8: 84.07,43.51 C40.2 IC10.5 v81.9,45.77 | 12.86,62.41 C52.2 IC13.5 v15.68,63.85 | 97.3,95.64 C48.2 IC12.5 v94.5,94.21 | 10.57,90.44 C68.2 IC17.5 v13.65,89.91 | 99.16,67.31 C60.2 IC15.5 v96.04,67.85 | 57.76,33.5 C56.2 IC14.5 v57.27,36.6 | 30.54,40.42 C76.2 IC19.5 v32.01,43.21 | 79.57,117.74 C72.2 IC18.5 v78.13,114.93 | 52.05,124.55 C64.2 IC16.5 v52.54,121.45 | IC3.1 26.1,25.2 C6.1 18.94,25.2 C5.2 | v18.29,26.28 v17.49,26.28 17.49,25.98 v17.89,25.58 | v17.89,25.58 18.29,25.98 v18.29,26.28 | v18.29,26.28 18.99,25.58 | 18.99,25.58 18.99,25.18 18.29,25.18 v17.89,25.58 | 18.99,25.58 19.38,25.2 19.82,25.2 | C44.2 IC11.5 27.04,112.93 v27.84,112.15 | C44.2
  Top 1: 19.87,29.42 C4.1 19.87,30.48 20.74,30.48 21.09,30.48 | 19.29,31.08 v18.89,31.48 | 20.99,29.68 v21.99,29.98 | 19.19,30.28 v18.89,30.58 | 17.99,30.58 v17.49,31.08 18.49,31.08
  Top 1.2: C3.2 19.87,29.42 | 21.56,29.42 21.12,29.42 20.99,29.68 v18.89,29.68 17.89,29.68 v17.49,30.08 v17.49,31.08 17.89,31.48 v18.89,31.48 | v20.69,31.28 v21.99,29.98 v20.69,29.98 | v20.69,31.28 19.29,31.08 | v20.69,29.98 19.19,30.28 | v18.89,30.58 17.99,30.58 | 18.49,31.08 v18.89,31.48 | v18.89,31.48 v20.69,31.28 | v20.69,29.98 20.74,30.48
  Bottom 0.7: v77.5,114.58 v78.12,114.21 v78.13,114.93 v77.5,114.58 | v93.78,94.25 v94.1,93.6 v94.5,94.21 v93.78,94.25 | v28.54,111.96 v27.84,112.15 v28.03,111.45 | v28.54,111.96 v28.03,111.45 | v28.43,108.55 v28.07,107.93 v28.79,107.93 v28.43,108.55 | v14.33,90.17 v13.65,89.91 v14.21,89.45 | v14.33,90.17 v14.21,89.45 | v16.07,64.46 v15.68,63.85 v16.4,63.82 | v16.07,64.46 v16.4,63.82 | v95.48,68.3 v95.36,67.59 v96.04,67.85 v95.48,68.3 | v81.9,45.77 v81.2,45.96 v81.71,46.46 | v81.71,46.46 v81.9,45.77 | v32.01,43.21 v31.97,43.94 v32.61,43.61 | v32.61,43.61 v32.01,43.21 | v57.53,37.27 v56.81,37.16 v57.27,36.6 v57.53,37.27 | v16.15,87.01 v16.22,86.29 v16.81,86.72 v16.15,87.01 | v52.28,120.77 v53,120.88 v52.54,121.45 v52.28,120.77 | v49.91,117.99 v50.49,117.57 v50.57,118.28 | v49.91,117.99 v50.57,118.28 | v73.99,113.66 v74.22,112.96 v74.7,113.5 | v73.99,113.66 v74.7,113.5 | v35.56,44.67 v36.27,44.52 v36.05,45.21 v35.56,44.67 | v19.33,62.93 v19.81,62.39 v20.03,63.08 v19.33,62.93 | v90.4,95.65 v90.18,94.96 v90.88,95.11 | v90.4,95.65 v90.88,95.11 | v93.59,71.35 v93,70.92 v93.66,70.63 | v93.59,71.35 v93.66,70.63 | v81.58,49.53 v81.94,50.15 v81.22,50.15 v81.58,49.53 | v59.23,40.45 v59.82,40.02 v59.16,39.73 | v59.16,39.73 v59.23,40.45 | v74.7,113.5 v77.5,114.58 | v73.99,113.66 v78.14,114.93 v78.13,114.21 v74.21,112.96 | v90.88,95.11 v93.78,94.25 | v90.4,95.65 v94.5,94.21 v94.11,93.6 v90.18,94.97 | v93.66,70.63 v95.48,68.3 | v93.59,71.35 v96.04,67.85 v95.36,67.59 v93,70.92 | v81.58,49.53 v81.71,46.46 | v81.9,45.77 81.94,50.18 v81.22,50.15 v81.2,45.95 | v57.53,37.27 v59.16,39.73 | v59.23,40.45 v56.81,37.15 v57.27,36.6 v59.82,40.02
  Bottom 0.7: v32.61,43.61 v35.56,44.67 | v32.01,43.21 v36.28,44.52 v36.05,45.21 v31.97,43.94 | v16.4,63.82 v19.33,62.93 | v16.07,64.46 v20.03,63.08 v19.81,62.39 v15.68,63.85 | v14.21,89.45 v16.15,87.01 | v14.33,90.17 v16.81,86.72 v16.22,86.29 v13.65,89.91 | v28.03,111.45 v28.43,108.55 | v28.54,111.96 v28.79,107.92 v28.07,107.93 v27.84,112.15 | v50.57,118.28 v52.28,120.77 | v49.91,117.99 v52.54,121.45 v53,120.88 v50.49,117.57 | v27.04,115.78 v26.84,115.03 v26.29,115.58 v27.04,115.78 | v10.93,92.42 v11.21,91.69 v10.44,91.82 v10.93,92.42 | v54.02,124.88 v53.41,124.39 v53.29,125.16 v54.02,124.88 | v81.35,116.84 v80.58,116.8 v80.93,117.49 v81.35,116.84 | v98.2,93.86 v97.55,94.28 v98.24,94.63 v98.2,93.86 | v98.91,65.37 v98.63,66.1 v99.4,65.98 v98.91,65.37 | v82.69,42.08 v82.89,42.83 v83.44,42.28 v82.69,42.08 | v55.82,33.14 v56.42,33.63 v56.55,32.86 v55.82,33.14 | v28.76,41.32 v29.53,41.36 v29.18,40.67 v28.76,41.32 | v11.98,64.22 v12.63,63.8 v11.94,63.44 v11.98,64.22
  Bottom 1.7: 37.29,34.66 D1.C 35.49,31.43 | 35.49,31.43 38.09,29.96 | 35.49,31.43 32.57,33.06
  pour Bottom (rank 2): 54.34,41.39 54.34,26.38 52.89,28.38 38.69,28.38 34.99,22.68 16.1,22.68 16.1,43.62 arc-42 2.49,78.88 arc-90 54.99,131.38 arc-90 107.49,78.88 arc-90 54.99,26.38 54.99,41.38 arc90 92.49,78.88 arc90 54.99,116.38 arc90 17.49,78.88 arc89
CODE_0  (via drill 0.35 pad 0.7)
  Top 0.3: U1.53 59.26,14.06 v63.82,9.51 64.19,9.13 68.74,4.58 68.74,3.01 JP3.7 | RN1.1 65.79,12.08 v65.79,11.38
  Bottom 0.3: v65.79,11.38 63.92,9.51 v63.82,9.51
CODE_1  (via drill 0.35 pad 0.7)
  Top 0.3: U1.54 59.72,14.57 v65.17,9.12 65.4,8.89 JP3.5 | RN1.2 66.59,12.08 v66.59,10.68
  Bottom 0.3: v66.59,10.68 65.17,9.27 v65.17,9.12
CODE_2  (via drill 0.35 pad 0.7)
  Top 0.3: U1.55 60.22,15.05 v66.42,8.86 66.69,8.58 68.79,6.48 JP3.3 | RN1.3 67.39,12.08 v67.39,9.83
  Bottom 0.3: v67.39,9.83 v66.42,8.86
CODE_3
  Top 0.3: U1.56 60.66,15.56 67.57,8.66 | 67.57,8.66 68.22,8.01 69.33,8.01 JP3.1 | RN1.4 68.17,9.27 67.57,8.66
GND  (via drill 0.35 pad 0.7)
  Top 0.3: v84.3,40.39 R30.1 | v9.78,63.1 R36.1 | v82.42,118.92 R46.1 | v101.17,64.89 R40.1 | v8.51,92.82 R44.1 | v56.13,30.76 R38.1 | v53.7,127.21 R42.1 | v25.36,117.44 R32.1 | v100.33,94.91 R34.1 | U1.16 48.07,21.4 v48.07,20.26 48.63,20.82 U1.15 | U1.47 55.13,10.95 v54.56,11.52 | v47.81,12.17 47.42,12.57 U1.31 | v42.21,11.62 42.21,10.67 42.91,10.67 42.91,9.82 Q1.GND1 | 20.81,3.94 20.74,3.88 20.74,3.45 | IC2.2 20.79,10.01 20.79,9.08 v20.49,8.78 | U1.4 54.14,22.92 C20.- | v26.59,38.74 26.79,39.18 R48.1
  Top 0.5: X2.5 20.81,3.94 21.45,3.94 21.49,3.98 | PROG.3 PROG.5 44.76,24.01 v45.39,23.38 44.79,22.78 43.54,22.78 | OC1.5 v76.99,28.48 | C20.- 57.59,24.67 C21.1 57.63,24.68 v58.69,24.68 | X2.GND4 X2.GND3 X2.GND1 17.64,9.07 v17.64,10.83 | v19.24,1.48 X2.GND2 17.57,4.06 17.69,4.18
  Top 0.61: 7,87.39 D57.A
  Top 0.7: v32.64,107.83 v32.84,107.08 v32.09,107.28 | v32.64,107.83 v32.09,107.28 | v32.64,107.83 31.74,108.73 31.19,108.73 | v32.09,107.28 31.19,108.18 31.19,108.73 | 31.19,108.73 32.29,107.63 32.34,107.63 | v21.25,67.04 v22.02,67 v21.6,66.35 | v21.25,67.04 v21.6,66.35 | v34.64,49.06 v35.29,49.49 v35.33,48.71 | v34.64,49.06 v35.33,48.71 | v55.95,42.92 v56.23,43.64 v56.71,43.04 | v55.95,42.92 v56.71,43.04 | v77.14,50.13 v76.94,50.88 v77.69,50.68 | v77.14,50.13 v77.69,50.68 | v89.66,68.54 v89.05,69.03 v89.78,69.3 | v89.66,68.54 v89.78,69.3 | v88.93,90.98 v88.16,91.02 v88.58,91.67 | v88.93,90.98 v88.58,91.67 | v75.53,109.02 v74.88,108.6 v74.84,109.38 | v75.53,109.02 v74.84,109.38 | v53.91,115.14 v53.63,114.41 v53.14,115.01 | v53.91,115.14 v53.14,115.01 | v21.6,66.35 20.54,65.78 R37.2 | v21.25,67.04 20.29,66.53 21.24,66.53 | v20.08,89.23 v20.68,88.74 v19.95,88.46 | v20.08,89.23 v19.95,88.46 | v19.95,88.46 18.99,88.63 R45.2 | v20.08,89.23 18.79,89.43 19.79,88.83 | v53.14,115.01 52.94,116.08 R43.2 | v53.91,115.14 53.74,116.08 53.54,115.48 | v74.84,109.38 75.24,110.18 R47.2 | v75.53,109.02 75.89,109.78 75.44,109.58 | v88.58,91.67 89.44,92.13 R35.2 | v88.93,90.98 90.04,91.53 88.99,91.48 | v89.78,69.3 90.59,69.18 R41.2 | v89.66,68.54 90.99,68.33 89.84,68.93 | v77.14,50.13 77.59,49.68 R31.2 | v77.69,50.68 78.54,49.83 77.69,50.13 | v56.71,43.04 56.84,42.28 R39.2 | v55.95,42.92 56.14,41.78 56.49,42.83 | v35.33,48.71 34.94,47.98 34.84,48.48 R49.2 | v34.64,49.06 34.19,48.18
  Top 0.8: IC10.2 78.55,49.06 R31.2 78.55,49.24 | 88.75,43.91 D22.A | v87.23,40.43 87.36,40.7 87.21,40.4 | v89.04,41.91 v89.02,41.91 | v87.52,42.65 87.48,42.64 | IC13.2 19.85,65.95 R37.2 20.02,65.89 | 11.8,57.83 D37.A 11.77,57.56 | v8.95,60.4 9.33,59.92 9.57,59.61 8.93,60.39 | v9.81,58.23 9.8,58.19 | v10.95,59.43 10.98,59.44 | IC12.2 90.31,92.11 R35.2 90.14,92.16 | 98.36,100.22 D32.A | C50.1 101.77,99.4 | C46.1 20.69,117.47 | 48.02,126.98 D52.A | C66.1 49.85,129.97 | C68.1 7.56,90.9 | 62.02,31.11 D42.A | C58.1 59.95,28.08 | 102.71,70.39 D47.A | C62.1 104.99,67.72 | 77.74,122.07 D62.A | C74.1 80.98,123.41 | 32.38,36.1 D69.A | C78.1 29.13,34.75 | C70.1 4.75,90.03 | 7.02,87.36 D57.A | v101.25,97.71 101.25,97.68 101.23,97.67 | v99.16,98.63 99.18,98.62 | v100.35,99.87 100.35,99.86 | v20.68,115.97 20.69,115.97 | v22.24,115.23 22.23,115.24 | v22.48,117.5 22.5,117.48 | v6.15,91.09 6.18,91.12 6.2,91.11 | v5.67,88.86 5.62,88.83 | v7.31,89.15 7.3,89.14 | v102.42,68.6 102.43,68.62 | v104.11,68.95 104.11,68.93 | v103.53,66.66 103.55,66.64 103.53,66.64 | v51.31,128.92 51.33,128.94 51.33,128.91 | v49.78,127.25 v49.79,127.26 | v48.98,128.78 48.98,128.76 | v60.83,29.32 60.83,29.29 | v58.5,29.14 58.48,29.11 58.48,29.14 | v60.03,30.8 60.01,30.79 | v30.55,35.26 30.55,35.22 | v30.77,36.93 30.78,36.91 | v28.54,36.47 28.55,36.45 28.56,36.47 | v79.34,121.23 79.34,121.25 | v79.56,122.96 v79.56,122.95 | v81.57,121.74 81.57,121.71 81.55,121.69 | 31.17,108.82 R33.2 | 31.17,108.64 R33.2 | IC17.2 18.31,89.2 R45.2 18.41,89.05 | IC15.2 91.43,68.56 R41.2 91.32,68.71 | IC14.2 56.56,41.24 R39.2 56.66,41.38 | IC19.2 34.12,47.39 R49.2 34.29,47.45 | 75.82,110.71 R47.2 75.99,110.77 IC18.2 | IC16.2 53.25,116.81 R43.2 53.14,116.67
  Top 0.8: C6.2 18.67,20.38 C5.1 18.02,21.78 | v18.79,21.48 v20.79,21.48 | v20.79,21.48 21.39,21.48 | v20.79,21.48 v19.79,20.48 v18.79,21.48 | v18.79,21.48 18.5,21.78 | 18.5,21.78 18.02,21.78 | 18.02,21.78 18.81,20.98 21.19,20.98 | 18.5,21.78 21.59,21.78 | C7.1 22.78,18.27 v23.19,18.68 v24.09,18.68 | C8.- 24.33,18.45 v24.09,18.68 | v24.09,18.68 22.99,17.58 24.29,17.58 | v29.09,10.68 29.09,9.75 C9.1 29.02,9.68 C10.- 30.56,9.78 v31.59,9.78 | C11.1 35.65,11.68 | 35.65,11.68 C12.- 36.41,10.1 v36.69,10.18 | 35.65,11.68 36.08,11.68 | 36.08,11.68 36.4,11.68 v36.69,11.38 36.69,8.09 IC4.1 | 36.08,11.68 36.08,10.3 36.09,10.28 | 21.49,3.98 22.46,4.95 L2.2 23.27,4.73 C2.1 25.29,4.79 v25.29,5.78 | 21.45,3.94 20.99,3.48 v20.99,3.18 | IC11.2 31.17,108.82 | 31.17,108.82 R33.2 | 31.19,108.73 R33.2
  Top 1: 22.07,35.5 23.19,34.38 23.19,34.28 23.99,35.08 v23.99,38.28 | 22.07,35.5 C4.2 | 20.89,38.28 v22.24,38.28 | v22.24,38.28 v23.99,38.28 | v23.99,38.28 23.89,38.28 v23.09,38.98 | v23.09,38.98 v23.79,39.78 v22.24,39.78 | v22.24,39.78 v20.49,39.78 v20.49,38.28 20.89,38.28 | v22.24,38.28 v21.34,38.98 | 20.89,38.28 v22.24,39.78 | v22.24,39.78 22.29,38.38 v22.24,38.28 | C4.2 19.87,37.56 v21.34,38.98 | 22.07,35.5 23.99,37.42 v23.99,38.28 | v23.99,38.28 23.29,38.98 v23.09,38.98 | v23.09,38.98 v21.34,38.98 | v21.34,38.98 20.69,38.38 20.69,36.08 20.89,36.28 22.09,36.28 23.19,37.38 | 23.19,37.38 23.19,37.48 | 23.19,37.48 23.19,37.88 22.89,37.58 21.49,37.58 21.39,37.48 21.39,36.88 21.59,37.08 22.29,37.08 | v23.99,38.28 23.19,37.48 | 23.19,37.38 23.19,35.08 | C4.2 19.87,35.08 23.89,35.08
  Top 1.2: C40.1 87.21,40.4 C42.1 | C40.1 87.48,42.64 88.75,43.91 | D22.A 89.02,43.97 v89.02,41.91 89.02,40.38 | 11.8,57.83 10.98,59.44 C52.1 8.93,60.39 C54.1 | 11.77,57.56 9.8,58.19 8.35,58.67 | 98.36,100.22 99.18,98.62 C48.1 101.23,97.67 C50.1 100.29,97.98 99.59,99.38 100.59,99.18 | 101.77,99.4 100.35,99.86 98.22,100.56 | D27.A 20.96,113.97 22.23,115.24 C44.1 22.5,117.48 C46.1 22.64,116.63 21.39,115.08 21.24,116.58 | 20.69,117.47 20.69,115.97 20.69,113.55 | 48.02,126.98 v49.79,127.26 C64.1 51.33,128.91 C66.1 50.84,127.98 48.89,127.68 49.74,128.78 | 49.85,129.97 48.98,128.76 47.55,126.8 | C56.1 60.01,30.79 62.02,31.11 | C56.1 58.48,29.14 C58.1 | 59.95,28.08 60.83,29.29 62.25,31.25 | 102.71,70.39 102.43,68.62 C60.1 103.53,66.64 C62.1 102.89,67.43 103.04,69.33 103.94,68.23 | 104.99,67.72 104.11,68.93 102.79,70.75 | 77.74,122.07 79.34,121.25 C72.1 81.55,121.69 C74.1 80.89,121.38 79.24,122.03 80.19,122.53 | 80.98,123.41 v79.56,122.95 77.42,122.25 | C76.1 30.78,36.91 32.38,36.1 | C76.1 28.56,36.47 C78.1 | 29.13,34.75 30.55,35.22 32.86,35.97 | 4.75,90.03 5.62,88.83 6.11,88.16 | 6.11,88.16 6.73,87.3 | 7.02,87.36 7.3,89.14 C68.1 6.2,91.11 C70.1 | C3.1 23.19,32.2 23.19,34.28 | C40.1 88.54,42.73 88.54,41.43 87.24,40.98 | C56.1 60.84,30.33 59.79,29.28 58.89,29.58 | C76.1 30.99,36.13 29.59,35.78 29.24,36.33 | 9.33,59.92 10.19,59.43 10.74,58.43 9.14,59.23 | 6.11,88.16 6.04,90.48 6.94,90.33 6.69,88.73
  Bottom 0.3: 48.07,19.16 C25.1 | 48.07,19.08 C25.1 | 48.2,19.03 C25.1 | v50.12,16.08 C13.1
  Bottom 0.5: v48.07,20.26 48.07,19.16 | v48.2,18.23 48.2,19.03 | D5.C 24.89,17.11 D6.C 27.73,17.09 v28.97,17.09 | TP6.TP 32.49,17.11 D8.C v31.37,17.09 v31.37,17.08 D7.C | D4.C 30.19,19.14 D7.C v28.97,17.09 | C22.2 v52.39,16.24 v52.39,16.23 | v28.97,17.09 v28.97,17.08
  Bottom 0.7: v32.84,107.08 v32.09,107.28 v32.64,107.83 v32.84,107.08 | v22.02,67 v21.6,66.35 v21.25,67.04 v22.02,67 | v35.29,49.49 v35.33,48.71 v34.64,49.06 v35.29,49.49 | v56.23,43.64 v56.71,43.04 v55.95,42.92 v56.23,43.64 | v76.94,50.88 v77.69,50.68 v77.14,50.13 v76.94,50.88 | v89.05,69.03 v89.78,69.3 v89.66,68.54 v89.05,69.03 | v88.16,91.02 v88.58,91.67 v88.93,90.98 v88.16,91.02 | v74.88,108.6 v74.84,109.38 v75.53,109.02 v74.88,108.6 | v53.63,114.41 v53.14,115.01 v53.91,115.14 v53.63,114.41 | v20.68,88.74 v19.95,88.46 v20.08,89.23 v20.68,88.74
  Bottom 1: PJ1.2 v21.34,38.98
  Bottom 3: PJ1.2 PJ1.3
  other vias: 41.96,5.97 46.21,10.42 47.26,6.92 27.49,38.08 28.09,39.38 20.49,36.58 21.09,35.28 21.69,36.58 22.89,36.58 22.39,35.28 23.69,35.28 50.21,128.42 80.27,121.94 100.5,98.56 103.47,68 87.87,41.45 59.6,29.64 29.79,36.13 9.65,59.55 6.35,89.79 21.93,116.47 57.04,28.98 58.74,27.18 65.19,26.93 67.99,28.96 70.22,33.38 72.69,32.36 73.52,35.86 75.89,34.71 74.92,40.26 78.84,36.58 80.62,38.91 78.82,40.36 77.22,40.48 76.22,42.96 73.82,45.13 75.27,49.21 76.34,54.53 80.24,55.51 80.07,58.61 85.42,61.11 83.92,63.73 86.69,65.01 85.67,69.28 90.09,76.11 94.52,80.13 97.82,85.46 100.24,84.51 103.17,86.38 102.29,88.73 100.67,91.11 98.67,89.66 89.57,80.68 71.97,48.91 96.12,88.26 92.52,86.26 88.99,89.16 85.04,90.33 84.87,97.31 80.54,100.56 81.22,104.23 76.44,107.93 68.24,108.18 65.47,112.13 64.47,110.08 59.77,113.73 45.54,114.43 42.59,113.38 38.72,118.68 34.57,118.36 34.74,120.96 33.02,122.78 30.27,121.38 28.97,118.86 31.24,117.28 32.57,117.31 36.07,112.28 34.29,108.91 35.62,106.31 31.04,104.33 30.47,99.81 27.14,99.18 25.97,93.56 23.27,92.61 24.17,86.98 20.72,83.41 18.27,78.21 14.69,78.06 11.02,71.86 8.89,73.93 6.24,72.56 7.44,69.58 9.42,67.23 11.44,68.53 12.52,102.26 14.47,100.93 10.39,96.21 10.37,98.86 10.17,100.98 13.97,98.43 13.27,96.03 11.19,105.76 8.62,105.93 13.14,112.11 18.19,113.28 16.42,115.23 23.62,118.66 23.57,121.73 28.17,122.71 30.84,126.43 36.47,126.41 41.74,130.13 45.57,127.96 53.22,128.38 57.62,128.66 60.44,127.66 62.49,127.61 63.12,125.23 61.79,123.51 60.37,123.73 57.32,126.63 68.37,127.93 67.67,130.21 74.39,128.31 76.34,124.23 83.02,120.58 86.27,120.88 86.74,117.08 90.72,116.28 91.94,111.56 99.27,107.68 98.39,103.01 101.94,96.31 105.62,93.23 103.89,89.26 107.47,83.76 105.57,81.13 107.67,75.48 104.29,72.73 102.52,65.21 100.97,60.11 99.54,58.61 95.47,59.33 95.39,56.31 99.12,61.66 96.59,61.63 96.47,53.38 98.89,56.36 99.02,51.36 96.17,45.66 91.14,44.63 85.64,39.38 82.64,35.28 80.42,36.76 77.89,32.91 70.97,35.03 64.39,34.78 64.84,32.51 59.49,33.73 52.14,29.88 52.24,32.08 51.69,33.71 50.22,34.88 48.99,34.18 47.32,34.56 46.22,33.51 48.49,30.26 49.04,28.43 64.59,30.46 44.74,30.63 41.39,30.48 45.32,28.13 38.77,28.26 20.19,43.83 24.99,42.16 25.97,45.08 24.07,46.26 22.39,47.38 20.12,46.06 21.29,41.61 43.19,36.23 45.14,38.11 42.02,42.66 44.74,46.88 44.82,52.93 49.04,56.48 52.37,66.86 51.69,61.56 59.14,68.96 57.49,66.26 65.14,71.13 66.09,78.86 69.34,84.21 65.32,84.78 73.19,87.81 80.44,88.78 83.02,91.88 87.77,99.88 84.14,103.88 87.42,106.93 86.12,111.21 84.64,112.13 89.49,111.96 87.69,115.41 84.89,115.93 89.94,113.78 57.47,91.16 49.99,90.28 44.97,86.31 43.17,79.43 45.54,71.76 61.94,88.96 25.39,55.96 24.22,100.18 26.92,67.28 11.29,49.11
  pour Route2: 9.03,-7.07 9.03,32.92 arc-270 100.95,32.92 100.89,35.13 77.99,35.13 77.99,8.63 88.09,8.63 88.09,-7.07
  pour Top: 48.56,11.67 48.61,12.57 44.66,12.57 42.61,12.62 41.41,11.22 40.51,11.22 38.26,8.97 38.26,8.02 43.61,2.67 45.01,2.67 48.61,6.27 48.61,10.62
  pour Route3 (rank 2): 54.99,133.88 arc-90 109.99,78.88 arc-90 54.99,23.88 arc-90 -0.01,78.88 arc-90
GND-USB  (via drill 0.35 pad 0.7)
  Top 0.3: IC5.20 84.85,25.63 84.29,26.18 v84.29,26.73 | IC5.4 84.35,19.78 84.64,19.48 84.64,18.4 C29.1 | IC5.24 82.65,25.13 v81.59,25.13 81.59,24.18 81.89,23.89 IC5.26 | IC5.17 87.1,25.69 C27.-
  Top 0.5: 89.14,15.03 88.49,15.03 87.48,14.02 L1.2 84.54,14.02 C1.1 | 89.14,15.03 X1.5 | v91.27,25.63 TP7.TP | v89.74,18.23 89.74,19.39 IC1.2 | v89.14,15.83 89.14,15.03 | C27.- 87.1,28.44 C26.1 87.04,28.49 v87.04,29.23 | 88.14,26.33 88.19,26.38 C28.1 | v85.64,18.28 84.59,18.28 C29.1 | 88.38,26.63 C28.1 | C28.1 88.39,26.64 v88.39,27.48 | OC2.5 v83.19,13.83 84.44,13.83 | X1.GND1 X1.GND3 X1.GND4 X1.GND2 92.54,17.54 v92.54,19.28 | v90.69,9.83 92.39,9.83 92.49,9.93
  pour Route2: 79.29,9.93 79.29,33.83 94.99,33.83 94.99,8.18 90.69,8.18 88.64,9.93
LED0
  Top 0.3: U1.42 52.64,7.43 54.39,5.68 55.21,5.68 JP8.1
  Bottom 0.5: D11.C 56.97,4 JP8.1
LED1
  Top 0.3: U1.41 52.14,7.09 54.04,5.18 55.04,5.18 55.69,4.53 55.69,2.66 JP8.2
  Bottom 0.5: D12.C 55.67,2.69 JP8.2
LED2
  Top 0.3: U1.40 51.63,6.73 JP8.3
  Bottom 0.5: D13.C 54.4,3.98 JP8.3
LED_WHITE8  (via drill 0.35 pad 0.7)
  Top 0.3: 34.74,93.93 v34.74,93.43 | 30.41,75.2 v30.41,74.86
  Top 0.7: v30.41,74.86 v31.33,74.86 v30.83,75.56 v29.91,75.56 v29.49,74.86 v30.41,74.86 | v30.41,74.86 30.41,75.21 | v34.74,93.43 v35.39,92.78 v35.54,93.63 v34.89,94.28 v34.09,94.08 v34.74,93.43 | v34.74,93.43 34.99,93.68
  Top 0.8: D59.A
  Top 1.2: D58.C 34.74,93.93 | D59.A 30.41,75.2
  Bottom 0.3: 35.23,93.43 v34.74,93.43 | 30.75,75.2 v30.41,74.86
  Bottom 0.7: v30.41,74.86 v31.33,74.86 v30.83,75.56 v29.91,75.56 v29.49,74.86 v30.41,74.86 | v30.41,74.86 30.41,75.21 | v34.74,93.43 v35.39,92.78 v35.54,93.63 v34.89,94.28 v34.09,94.08 v34.74,93.43 | v34.74,93.43 34.99,93.68
  Bottom 1.2: 35.23,93.43 39.91,88.76 40.53,85.8 arc32 39.1,77 37.3,75.2 30.75,75.2
MCU_UART1_RXD
  Top 0.5: OC1.4 75.15,29.78 74.04,29.78 72.86,28.6 JP1.3 74.95,25.22 R21.2
MCU_UART1_TXD
  Top 0.5: JP1.1 77.07,20.56 R24.1
MCU_UART2_RXD  (via drill 0.35 pad 0.7)
  Top 0.3: U1.59 62.72,17.06 v63.89,15.88 | v78.99,5.48 81.43,7.92 JP2.2
  Bottom 0.3: v63.89,15.88 69.39,10.38 73.59,10.38 75.04,8.93 75.04,7.13 76.69,5.48 v78.99,5.48
MCU_UART2_TXD  (via drill 0.35 pad 0.7)
  Top 0.3: U1.60 63.21,17.57 v63.89,16.88
  Bottom 0.3: v63.89,16.88 67.64,13.13 73.54,13.13 75.74,10.93 75.74,7.58 77.09,6.23 83.47,6.23 JP2.1 85.23,8
N$1
  Top 0.5: IC19.1 33.77,44.29
  Top 0.8: 33.77,44.29 36.16,43.07 C77.1
  Top 1.2: C77.1 37.32,42.51 38.54,42.91 D68.C
N$2
  Top 1.2: D67.1 39.95,46.7 40.15,46.08 D68.A
N$3
  Top 0.3: IC5.18 85.85,25.41 86.22,25.78 86.22,30.51 R10.1
N$4
  Top 0.78: IC19.6 32.23,41.48
  Top 0.8: 32.23,41.48 32.5,40.57 D69.C | 42.56,38.86 L29.1
  Top 1.2: D69.C C77.2 38.25,39.79 39.76,40.29 42.56,38.86
N$5
  Top 0.5: 27.34,33.63 27.36,33.62
  Top 0.8: 31.81,33.34 C78.2 | 38.87,31.62 L29.2
  Top 1.2: 27.36,33.62 30.44,32.06 31.3,32.34 31.81,33.34 | C78.2 33.85,32.32 36.07,33.04 38.87,31.62 | D70.A 43.23,58.82 43.23,55.98 38.71,51.47 37.13,51.43 32.83,53.61 28.86,52.21 26.53,47.63 C79.1 24.99,39.26 26.11,35.81 26.74,35.48 27.34,33.63
N$6
  Top 1.2: D70.C 37.21,65.05 arc-31 32.72,76.01 D71.A
N$7
  Top 1.2: D71.C 32.72,81.76 arc-31 37.21,92.71 D72.A
N$8
  Top 1.2: D72.C 41.16,96.67 arc-31 52.12,101.16 D73.A
N$9  (via drill 0.35 pad 0.7)
  Top 0.3: IC5.22 83.85,25.33 83.29,25.88 v82.69,25.88 | v91.85,27.54 v91.84,27.53
  Top 0.5: D9.C v91.85,27.54
  Bottom 0.5: v91.84,27.53 90.99,26.68 85.84,26.68 85.04,25.88 v82.69,25.88
N$10
  Top 0.3: U1.32 45.5,12.06 44.36,10.92 R8.2 42.08,7.27 40.78,7.27 Q1.1 40.58,7.54 C23.1
N$11
  Top 0.3: U1.33 48.12,9.43 47.04,8.35 R8.1 44.86,7.65 44.86,6.82 45.1,6.58 Q1.3 46.18,5.27 C24.1
N$12
  Bottom 0.5: D11.A 58.29,7.65 R14.1
N$13
  Top 0.5: X1.1 86.84,12.44 L1.1
N$14  (via drill 0.35 pad 0.7)
  Top 0.3: X1.2 88.79,13.09 v88.44,13.43 | v88.44,17.78 88.79,18.13 88.79,19.39 IC1.1
  Bottom 0.3: v88.44,13.43 v88.44,17.78
N$15
  Top 0.3: 90.74,19.36 IC1.3 90.7,16.68 90.94,16.43 90.94,14.08 90.6,13.74 X1.3
N$16
  Bottom 0.5: R3.1 30.21,22.08 D4.A
N$17
  Top 0.5: X2.1 20.76,6.89 21.51,6.89 21.49,6.88 21.49,6.74
  Top 0.8: L2.1 22.86,6.74 21.49,6.74 20.9,6.74
N$18
  Bottom 0.5: D5.A R4.1
N$19  (via drill 0.35 pad 0.7)
  Top 0.3: IC5.21 84.35,25.48 v83.04,26.78
  Top 0.5: v88.29,28.33 88.31,28.32 D10.C
  Bottom 0.5: v83.04,26.78 84.59,28.33 v88.29,28.33
N$20
  Top 0.7: IC19.3 31.79,45.28
  Top 0.8: 29.01,46.97 C79.2 29.34,46.53 31.79,45.28
  Top 1.2: 29.01,46.97 R49.1 31.11,51.05 33.36,51.8 37.7,49.61 39.37,49.61 45.29,55.54 45.29,68.83 arc-150 57.96,92.62 59.57,94.24 59.57,100.35 58.54,101.38 D73.C
N$21
  Top 0.5: R12.1 D10.A
N$22
  Top 0.5: R11.2 D9.A
N$23  (via drill 0.35 pad 0.7)
  Top 0.3: IC5.11 v87.79,21.89 v87.79,21.88
  Top 0.5: v91.59,21.88 92.26,21.88 R13.1
  Bottom 0.5: v87.79,21.88 v91.59,21.88
N$24
  Top 0.5: IC14.1 58.19,38.54
  Top 0.8: 58.19,38.54 60.75,38.94 C57.1
  Top 1.2: C57.1 62.01,39.17 62.77,40.21 D41.C
N$25
  Top 0.5: IC18.1 76.24,113.92
  Top 0.8: 76.24,113.92 73.95,115.09 C73.1
  Top 1.2: C73.1 72.79,115.65 71.58,115.25 D61.C
N$26
  Top 0.3: X2.2 19.59,5.89 19.09,6.38 19.09,8.48 19.89,9.28 IC2.1
N$27  (via drill 0.35 pad 0.7)
  Top 0.3: X2.3 21.25,5.24 v21.69,5.68 | v21.69,8.88 21.79,8.98 IC2.3
  Bottom 0.3: v21.69,5.68 v21.69,8.88
N$28
  Top 1.2: D60.1 70.17,111.46 69.96,112.09 D61.A
N$29
  Top 0.78: IC18.6 77.89,116.69
  Top 0.8: 77.89,116.69 77.62,117.59 D62.C | 67.55,119.3 L28.1
  Top 1.2: D62.C C73.2 71.75,118.43 70.23,117.93 67.55,119.3
N$30
  Top 0.8: 78.31,124.82 C74.2 | 71.24,126.54 L28.2
  Top 1.2: 78.31,124.82 78.81,125.82 79.67,126.1 83.4,124.19 85.12,118.9 C75.1 83.66,110.44 81.3,105.74 77.03,104.37 73.08,106.35 71.32,106.35 66.76,101.78 66.76,98.93 D63.A | C74.2 76.14,125.9 73.92,125.18 71.24,126.54
N$31
  Top 1.2: D64.A 77.26,81.76 arc31 72.77,92.71 D63.C
N$32
  Top 1.2: D65.A 72.77,65.05 arc31 77.26,76.01 D64.C
N$33
  Top 1.2: D66.A 57.87,56.61 arc31 68.82,61.1 D65.C
N$34
  Top 0.7: IC18.3 78.39,112.83
  Top 0.8: 79.97,108.79 R47.1 | 78.39,112.83 80.69,111.7 C75.2
  Top 1.2: C75.2 79.97,108.79 | R47.1 79.06,107.26 76.35,106.33 72.14,108.43 70.35,108.43 64.69,102.77 64.69,88.94 arc-148 51.76,65.23 50.14,63.62 50.14,57.51 51.27,56.39 D66.C
N$35
  Top 1.2: D40.1 61.68,44.11 62.21,43.72 D41.A
N$36
  Bottom 0.5: R15.1 56.38,8.72 55.67,8.01 D12.A
N$37
  Bottom 0.5: R16.1 57.18,10.82 54.4,8.04 D13.A
N$38
  Top 0.78: IC14.6 58.49,35.38
  Top 0.8: 58.49,35.38 59.4,34.66 61.29,34.96 D42.C | 68.4,39.3 L24.1
  Top 1.2: D42.C C57.2 64.49,37.54 65.43,38.83 68.4,39.3
N$39  (via drill 0.35 pad 0.7)
  Top 0.7: v35.69,54.33 v35.04,54.98 v34.89,54.13 v35.54,53.48 v36.34,53.68 v35.69,54.33 | v35.69,54.33 35.44,54.08 | v45.44,43.23 v44.79,43.88 v44.64,43.03 v45.29,42.38 v46.09,42.58 v45.44,43.23 | v45.44,43.23 45.19,42.98
  Top 0.8: 62.95,28.51 C58.2 | 69.67,31.27 L24.2 | C59.1 53,34.76
  Top 1.2: C59.1 53.95,29.3 58.45,26.02 62.59,26.68 63.12,27.4 62.95,28.51 | C58.2 65.33,28.91 66.7,30.8 69.67,31.27 | D43.A 35.69,54.38 v35.69,54.33 | 53,34.76 52.07,34.76 48.89,37.93 48.89,39.28 45.19,42.98
  Bottom 0.7: v35.69,54.33 v35.04,54.98 v34.89,54.13 v35.54,53.48 v36.34,53.68 v35.69,54.33 | v35.69,54.33 35.44,54.08 | v45.44,43.23 v44.79,43.88 v44.64,43.03 v45.29,42.38 v46.09,42.58 v45.44,43.23 | v45.44,43.23 45.19,42.98
  Bottom 1.2: 35.44,54.08 35.44,52.78 45.19,43.03 45.19,42.98
N$40  (via drill 0.35 pad 0.7)
  Top 0.3: 58.68,54.1 v59.02,54.1 | 39.85,58.53 v40.34,58.53
  Top 0.7: v59.02,54.1 v59.02,55.02 v58.31,54.52 v58.31,53.6 v59.02,53.18 v59.02,54.1 | v59.02,54.1 58.67,54.1 | v40.34,58.53 v40.99,59.18 v40.14,59.33 v39.49,58.68 v39.69,57.88 v40.34,58.53 | v40.34,58.53 40.09,58.78
  Top 0.8: D44.A
  Top 1.2: D44.A 58.68,54.1 | D43.C 39.85,58.53
  Bottom 0.3: 58.68,54.1 v59.02,54.1 | 40.65,59.33 v40.14,59.33
  Bottom 0.7: v59.02,54.1 v59.02,55.02 v58.31,54.52 v58.31,53.6 v59.02,53.18 v59.02,54.1 | v59.02,54.1 58.67,54.1 | v40.34,58.53 v40.99,59.18 v40.14,59.33 v39.49,58.68 v39.69,57.88 v40.34,58.53 | v40.34,58.53 40.09,58.78
  Bottom 1.2: 58.68,54.1 58.68,61.19 56.88,62.99 arc-32 48.08,64.43 45.11,63.8 40.65,59.33
N$41
  Top 0.5: IC15.1 94.49,69.25
  Top 0.8: 94.49,69.25 94.91,71.83 C61.1
  Top 1.2: C61.1 95.08,73.11 94.33,74.14 D46.C
N$42
  Top 1.2: D45.1 90.28,74.31 90.81,74.7 D46.A
N$43
  Top 0.7: IC14.3 55.94,38.18
  Top 0.8: 52.18,40.5 R39.1 52.12,40.73 | 55.94,38.18 53.24,37.68 C59.2
  Top 1.2: C59.2 52.18,40.5 | D44.C 58.68,47.01 57.6,45.93 55.62,45.93 52.12,42.42 52.12,40.73
N$44
  Top 0.78: IC15.6 97.58,68.58
  Top 0.8: 97.58,68.58 98.42,69.12 D47.C | 96.93,79.22 L25.1
  Top 1.2: D47.C C61.2 97.4,74.96 96.46,76.25 96.93,79.22
N$45
  Top 0.8: 105.51,70.7 C62.2 | 104.96,77.95 L25.2
  Top 1.2: 105.51,70.7 106.61,70.53 107.14,69.8 106.48,65.66 101.98,62.39 C63.1 94.07,60.9 93.14,59.96 92.96,59.78 79.3,59.78 D48.A | C62.2 105.9,73.34 104.53,75.23 104.96,77.95
N$46  (via drill 0.35 pad 0.7)
  Top 0.3: 79.66,82.57 v79.3,82.21 | 74.44,64.64 v74.44,65.13
  Top 0.7: v79.73,82.91 v78.81,82.91 v79.3,82.21 v80.22,82.21 v80.65,82.91 v79.73,82.91 | v79.73,82.91 79.73,82.56 | v75.09,64.48 v74.44,65.13 v74.29,64.28 v74.94,63.63 v75.74,63.83 v75.09,64.48 | v75.09,64.48 74.84,64.23
  Top 0.8: D49.A
  Top 1.2: D49.A 79.66,82.57 | D48.C 74.44,64.64
  Bottom 0.3: 79.73,82.58 v79.73,82.91 | 74.94,64.14 v74.94,63.63
  Bottom 0.7: v79.73,82.91 v78.81,82.91 v79.3,82.21 v80.22,82.21 v80.65,82.91 v79.73,82.91 | v79.73,82.91 79.73,82.56 | v75.09,64.48 v74.44,65.13 v74.29,64.28 v74.94,63.63 v75.74,63.83 v75.09,64.48 | v75.09,64.48 74.84,64.23
  Bottom 1.2: 79.73,82.58 72.52,82.58 70.89,80.95 arc-33 69.36,71.88 70.08,69.01 74.94,64.14
N$47  (via drill 0.35 pad 0.7)
  Top 0.3: U1.7 | U1.7 v52.64,19.88
  Bottom 0.3: 52.64,19.21 C22.1
  Bottom 0.5: v52.64,19.88 52.64,19.21
N$48
  Top 0.3: IC2.4 22.42,12.36 22.79,11.98 22.79,11.68 23.09,11.38 23.75,11.38 R2.1
N$49
  Top 0.3: 19.89,11.99 IC2.6 19.89,11.49 20.19,11.18 22.29,11.18 22.59,10.88 22.59,9.38 22.99,8.98 23.77,8.98 R1.1
N$50  (via drill 0.35 pad 0.7)
  Top 0.7: v86.58,83.49 v87.29,83.06 v87.29,82.14 v86.58,81.65 | v86.58,82.57 v86.58,81.65 | v86.58,83.49 v86.58,82.57 | v86.58,82.57 86.94,82.57 | v87.56,66.85 v87.56,65.93 v88.27,66.42 v88.27,67.34 v87.56,67.77 v87.56,66.85 | v87.56,66.85 87.92,66.85 87.92,66.16 88.19,65.88 | v86.58,83.49 86.58,83.43 85.69,83.43 | v86.58,81.65 86.58,81.63 85.69,81.63 | v86.58,83.49 v86.58,83.48 85.54,83.48 | IC15.3 94.14,66.98
  Top 0.8: 90.78,64.16 R41.1 | 94.14,66.98 93.74,64.38 C63.2
  Top 1.2: C63.2 90.78,64.16 89.91,64.16 88.19,65.88 | D49.C 85.44,82.57 v86.58,82.57
  Bottom 0.7: v86.58,82.57 v86.58,81.65 v87.29,82.14 v87.29,83.06 v86.58,83.49 v86.58,82.57 | v86.58,82.57 86.94,82.57 | v87.56,66.85 v87.56,65.93 v88.27,66.42 v88.27,67.34 v87.56,67.77 v87.56,66.85 | v87.56,66.85 87.92,66.85
  Bottom 1.2: 86.94,82.57 87.94,81.56 87.94,66.87 87.92,66.85
N$51
  Top 0.5: IC16.1 51.61,119.52
  Top 0.8: 51.61,119.52 49.06,119.11 C65.1
  Top 1.2: C65.1 47.79,118.88 47.04,117.84 D51.C
N$52
  Top 1.2: D50.1 48.13,113.95 47.6,114.33 D51.A
N$53
  Top 0.78: IC16.6 51.32,122.74
  Top 0.8: 51.32,122.74 50.55,123.29 D52.C | 41.4,118.75 L26.1
  Top 1.2: D52.C C65.2 45.19,120.49 44.25,119.2 41.4,118.75
N$54  (via drill 0.35 pad 0.7)
  Top 0.3: 74.93,104.03 74.93,104.02 74.64,103.73 | D53.A 73.93,103.02 v74.39,103.48
  Top 0.7: v74.39,103.48 v75.04,102.83 v75.19,103.68 v74.54,104.33 v73.74,104.13 v74.39,103.48 | v74.39,103.48 74.64,103.73 | v64.14,114.98 v64.79,114.33 v64.94,115.18 v64.29,115.83 v63.49,115.63 v64.14,114.98 | v64.14,114.98 64.39,115.23
  Top 0.8: 46.86,129.54 C66.2 | 40.17,126.91 L26.2 | D53.A 73.92,103.02
  Top 1.2: 46.86,129.54 46.69,130.65 47.21,131.37 51.35,132.03 55.86,128.76 C67.1 58.94,122.53 63.14,118.33 63.14,116.48 64.39,115.23 | C66.2 44.23,129.1 42.96,127.36 40.17,126.91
